(* Logix 5000 AddOnInstructionDefinition export Banner_QS18E_Param_v4; software revision 33.00 *)

TYPE Banner_IOL_Port_v4 :   // UDT that has all of the data items necessary to communicate with a specific Port on a IO-Link Master
STRUCT
   Port_Controlled : INT;   // Each bit represents a port on an IO-Link Master. Set to 1 to tell AOI to control that port.
   Port_Activate : INT;   // Each bit represents a port on an IO-Link Master. When ON that port will process any commands in queue.
   Port_Read : INT;   // Each bit represents a port on an IO-Link Master. Used to determine when device AOI has requested a Read command.
   Port_Write : INT;   // Each bit represents a port on an IO-Link Master. Used to determine when device AOI has requested a Write command.
   Port_RW_Complete : INT;   // Each bit represents a port on an IO-Link Master. Tells device AOI that Read or Write request has been completed.
   Port_Device_Read : INT;
   Data_Transfer : SINT[190];   // Array to transfer data from IO-Master to device AOIs.
END_STRUCT
END_TYPE

TYPE Banner_QS18E_1_v4 :   // Parameters for D, DV, LP, CV, and FP type sensors.
STRUCT
   Response_Speed : SINT;   // 0 = High Speed, 1 = Standard, 2 = Robust.
   Polarity_of_Pins_2_and_4 : SINT;   // 0 = Push Pull, 1 = PNP, 2 = NPN.
   Pin_2_Config : SINT;   // 0 = Deactivated, 1 = Pin 2 Emitter Enable, 2 = Pin 2 Emitter Disable, 3 = Remote Input, 4 = Detection Output, 5 = Complimentary Output, 6 = Normally Closed Health, 7 = Normally Open Health, 8 = Normally Closed Marginal, 9 = Normally Open Marginal.
   Process_Data_Input_Config : SINT;   // 0 = 5 and Signal, 1 = 5 and Count, 2 = 5 and Duration, 3 = 5 and Events per Minute.
   Marginal_Mode : SINT;   // 0 = Marginal Disabled, 1 = Marginal Auto, 2 = Marginal User.
   User_Marginal_Light : INT;   // 0 to 1000. User defined threshold.
   User_Marginal_Dark : INT;   // 0 to 1000. User defined threshold.
   LED_Power : SINT;   // 0 = Auto, 1 = Min Power, 2 = Power 2, 3 = Power 3, 4 = Power 4, 5 = Power 5, 6 = Max Power.
END_STRUCT
END_TYPE

TYPE Banner_QS18E_2_v4 :   // Parameters for EV and E type sensors
STRUCT
   Polarity_of_Pins_2_and_4 : SINT;   // 0 = Push Pull, 1 = PNP, 2 = NPN.
   Pin_2_Config : SINT;   // 0 = Deactivated, 1 = Pin 2 Emitter Enable, 2 = Pin 2 Emitter Disable, 3 = Remote Input, 4 = Detection Output, 5 = Complimentary Output, 6 = Normally Closed Health, 7 = Normally Open Health, 8 = Normally Closed Marginal, 9 = Normally Open Marginal.
   Frequency_Selection : SINT;   // 0 = High Speed, 1 = A, 2 = B, 3 = C.
   Power_Level : SINT;   // 0 to 5. Example: 5 = Power Level 5.
   Pushbutton_Lockout : SINT;   // 0 = Unlocked, 1 = Locked.
END_STRUCT
END_TYPE

TYPE Banner_QS18E_3_v4 :   // Parameters for RV and R type sensors
STRUCT
   Polarity_of_Pins_2_and_4 : SINT;   // 0 = Push Pull, 1 = PNP, 2 = NPN.
   Pin_2_Config : SINT;   // 0 = Deactivated, 1 = Pin 2 Emitter Enable, 2 = Pin 2 Emitter Disable, 3 = Remote Input, 4 = Detection Output, 5 = Complimentary Output, 6 = Normally Closed Health, 7 = Normally Open Health, 8 = Normally Closed Marginal, 9 = Normally Open Marginal.
   Process_Data_Input_Config : SINT;   // 0 = 5 and Signal, 1 = 5 and Count, 2 = 5 and Duration, 3 = 5 and Events per Minute.
   Marginal_Mode : SINT;   // 0 = Marginal Disabled, 1 = Marginal Auto, 2 = Marginal User.
   User_Marginal_Light : INT;   // 0 to 1000. User defined threshold.
   User_Marginal_Dark : INT;   // 0 to 1000. User defined threshold.
   Frequency_Selection : SINT;   // 0 = High Speed, 1 = A, 2 = B, 3 = C.
   IOL_Filter_Time : INT;   // Time in ms to average IOL process data measurement between updates.
   Gain : SINT;   // 0 = Auto - Teach, 1 = Auto - Run, 2 = Low Gain, 3 = Mid Gain, 4 = High Gain.
   Pushbutton_Lockout : SINT;   // 0 = Unlocked, 1 = Locked.
END_STRUCT
END_TYPE

TYPE Banner_QS18E_RD_v4 :   // UDT that stores the Write Data for a QS18E.
STRUCT
   Master_Cycle_Time : INT;
   Min_Cycle_Time : INT;
   M_Sequence_Capability : INT;
   IO_Link_Version_ID : INT;
   Process_Data_Input_Length : INT;
   Process_Data_Output_Length : INT;
   Combined_Vendor_ID : DINT;   // IO-Link Vendor ID
   Vendor_ID1 : INT;
   Vendor_ID2 : INT;
   Combined_Device_ID : DINT;   // IO-Link Device ID
   Device_ID1 : INT;
   Device_ID2 : INT;
   Device_ID3 : INT;
   Serial_Number : STRING;
   All_Time_Run_Time : DINT;   // Read only counter that tracks the total time sensor has been running since manufacture. Value in Hours.
   Quality_of_Health : INT;
   Normalized_Signal_Strength : INT;
   Quality_of_Teach : INT;
   Health_Lower_Limit : INT;
   Health_Upper_Limit : INT;
   SP2_Lower_Sensing_Threshold : INT;
   SP2_Upper_Sensing_Threshold : INT;
   SP1_Lower_Sensing_Threshold : INT;
   SP1_Upper_Sensing_Threshold : INT;
   Sensor_Operationl_Mode : INT;
   Output_Event_Count : DINT;
   Output_Event_Duration : DINT;
   Output_Event_Frequency : DINT;
   Active_Margninal_Light_Threshold : DINT;
   Active_Marginal_Dark_Threshold : DINT;
   Sigal : DINT;   // Only available for Sensor Type 3. Raw ADC Signal value.
END_STRUCT
END_TYPE

TYPE Banner_QS18E_v4 :   // All of the parameters for a QS18E.
STRUCT
   Initial_Global_Read : BOOL;   // Determines if all of the IO-Link data has been read into the PLC yet
   Command : INT;   // Value placed in here will activate a read or write to a specifc IO-Link Index
   Read_Data : Banner_QS18E_RD_v4;   // Read Only Data
   Write_Data : Banner_QS18E_WD_v4;   // Write Data
   Archive : Banner_QS18E_WD_v4;   // Archive Data
   Reset : BOOL;   // Resets AOI. This will force a complete parameter read of the sensor.
END_STRUCT
END_TYPE

TYPE Banner_QS18E_WD_v4 :   // UDT that stores the Write Data for a QS18E.
STRUCT
   System_Command : INT;   // See IODD file for list of commands that can be activated via the System Command interface
   Parameter_Access_Lock : SINT;   // Write access to all parameters is prohibited while value is 1. Only this parameter can be adjusted when value is 1.
   Data_Storage_Lock : SINT;   // Automatic data storage is disabled when this value is equal to 1. Read access is not affected.
   Local_Parameterization_Lock : SINT;   // Parameterization via local control elements on device is disabled.
   Local_User_Interface_Lock : SINT;   // Operation of local user interface is disabled.
   BDC1_Swithpoint_Logic : INT;   // 0 = Light Operate, 1 = Dark Operate
   BDC1_BDC_Mode : INT;   // 1 = 1-Pt BGS, 128 = 2-Pt, 129 = Dynamic, 130 = Window or FGS, 131 = Dual
   BDC1_Hysteresis : DINT;   // Should always be 0
   Marginal_Signal_Delay : DINT;   // 0 to 60000. Millisecond value
   User_Health_Setting : INT;   // 0 to 90
   Offset_Percent : INT;   // 0 = Min, 1 = 10%, 2 = 15%, 3 = 20%, 4 = 25%, 5 = 30%, 6 = 40%, 7 = 50%, 8 = 100%, 9 = 200%.
   Auto_Compensaton : INT;   // 0=Disabled, 1=Enabled
   Delay_Timer_2 : DINT;   // 0 to 90000 ms
   Delay_Timer_1 : DINT;   // 0 to 90000 ms
   Delay_Mode : INT;   // 0=Disabled, 1=On Off Delay, 2=On One Shot, 3=Off One Shot
   Resettable_Run_Time : DINT;
   Type_1_Data : Banner_QS18E_1_v4;   // Data for a D, DV, Lp, VC, or FP QS18E type sensor.
   Type_2_Data : Banner_QS18E_2_v4;   // Data for a E or EV QS18E type sensor.
   Type_3_Data : Banner_QS18E_3_v4;   // Data for a R or RV QS18E type sensor.
   All_Time_Run_Time_Event_Time : DINT;
   Resettable_Run_Time_Event_Time : DINT;
END_STRUCT
END_TYPE

ADD_ON_INSTRUCTION Banner_QS18E_Param_v4   (* revision 4.0, vendor Banner Engineering *)
// AOI to read and write parameter data to an IO-Link QS18E.
// Revision note:
// Updated for QS18 Emitter and Receiver.
VAR_IN_OUT
   QS18E : Banner_QS18E_v4; {required}
   Port_Data : Banner_IOL_Port_v4; {required}
END_VAR
VAR_INPUT
   Port : DINT; {required}
   Sensor_Type : DINT; {required}   // 1 = D, DV, LP, CV, & FP models, 2 = EV or E models, 3 = RV or R models.
END_VAR
VAR
   Local_Control : DINT; {access None}
   Global_Read_Command_Value : INT; {access None}
   Global_Write_Command_Value : INT; {access None}
   Command_Being_Processed : BOOL; {access None}
   Update_Archive : BOOL; {access None}
   Index_Write_Inprocess : INT; {access None}
   Index_Write_Control : INT; {access None}
   Inprocess_Index : DINT; {access None}
END_VAR

ROUTINE Logic   (* ladder *)
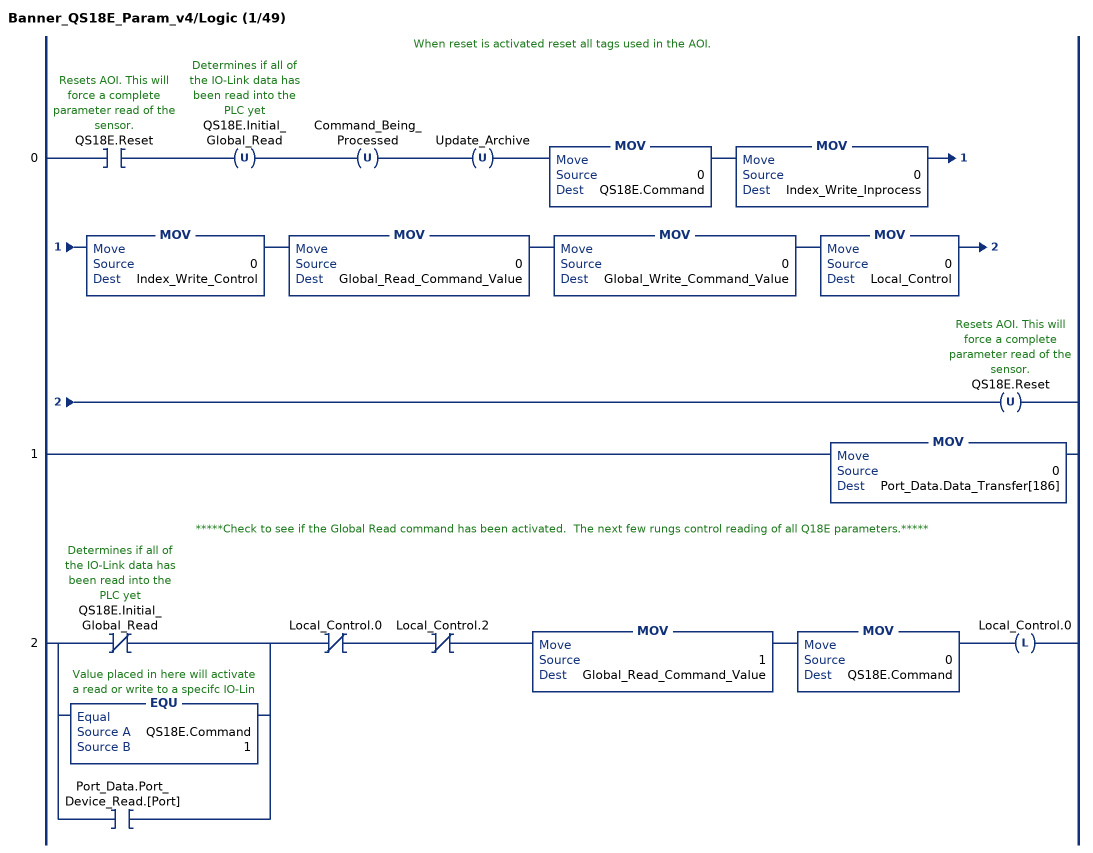
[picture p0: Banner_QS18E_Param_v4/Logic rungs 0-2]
   // When reset is activated reset all tags used in the AOI.
   0: XIC(QS18E.Reset)OTU(QS18E.Initial_Global_Read)OTU(Command_Being_Processed)OTU(Update_Archive)MOV(0,QS18E.Command)MOV(0,Index_Write_Inprocess)MOV(0,Index_Write_Control)MOV(0,Global_Read_Command_Value)MOV(0,Global_Write_Command_Value)MOV(0,Local_Control)OTU(QS18E.Reset);
   1: MOV(0,Port_Data.Data_Transfer[186]);
   // *****Check to see if the Global Read command has been activated.  The next few rungs control reading of all Q18E parameters.*****
   2: [XIO(QS18E.Initial_Global_Read) ,EQU(QS18E.Command,1) ,XIC(Port_Data.Port_Device_Read.[Port]) ]XIO(Local_Control.0)XIO(Local_Control.2)MOV(1,Global_Read_Command_Value)MOV(0,QS18E.Command)OTL(Local_Control.0);
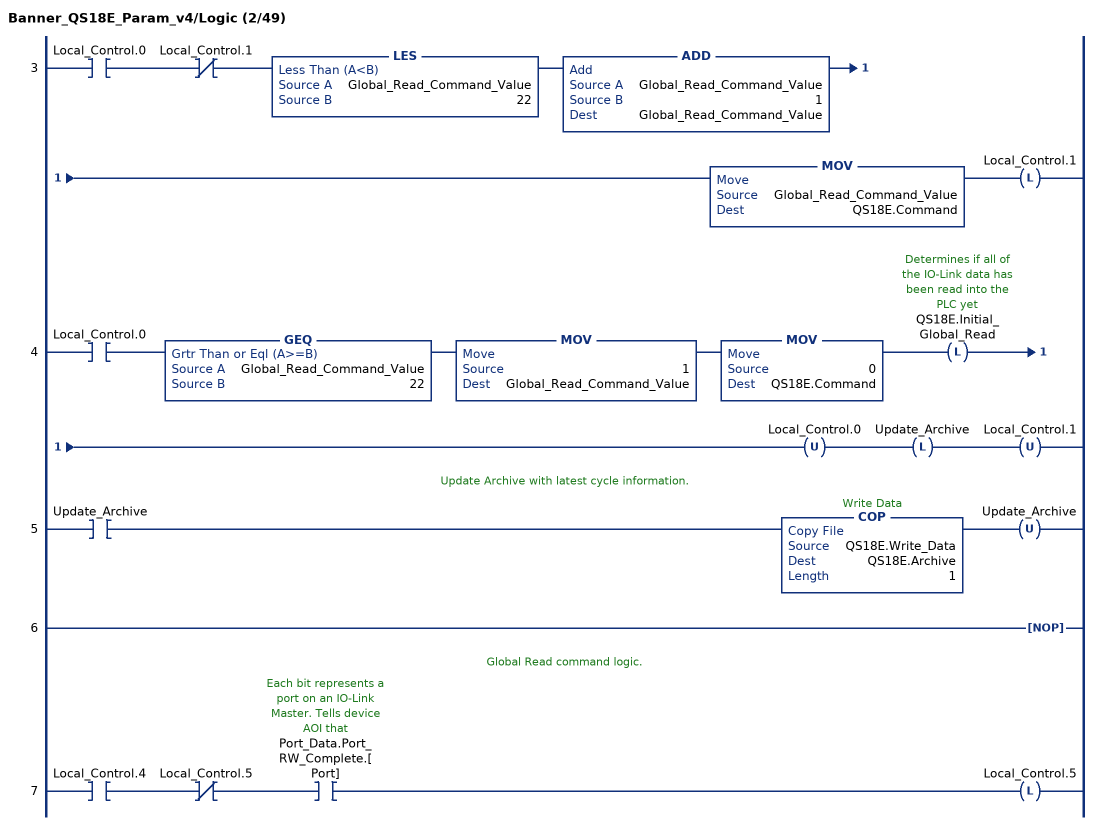
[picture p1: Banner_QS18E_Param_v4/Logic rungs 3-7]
   3: XIC(Local_Control.0)XIO(Local_Control.1)LES(Global_Read_Command_Value,22)ADD(Global_Read_Command_Value,1,Global_Read_Command_Value)MOV(Global_Read_Command_Value,QS18E.Command)OTL(Local_Control.1);
   4: XIC(Local_Control.0)GEQ(Global_Read_Command_Value,22)MOV(1,Global_Read_Command_Value)MOV(0,QS18E.Command)OTL(QS18E.Initial_Global_Read)OTU(Local_Control.0)OTL(Update_Archive)OTU(Local_Control.1);
   // Update Archive with latest cycle information.
   5: XIC(Update_Archive)COP(QS18E.Write_Data,QS18E.Archive,1)OTU(Update_Archive);
   6: NOP();
   // Global Read command logic.
   7: XIC(Local_Control.4)XIO(Local_Control.5)XIC(Port_Data.Port_RW_Complete.[Port])OTL(Local_Control.5);
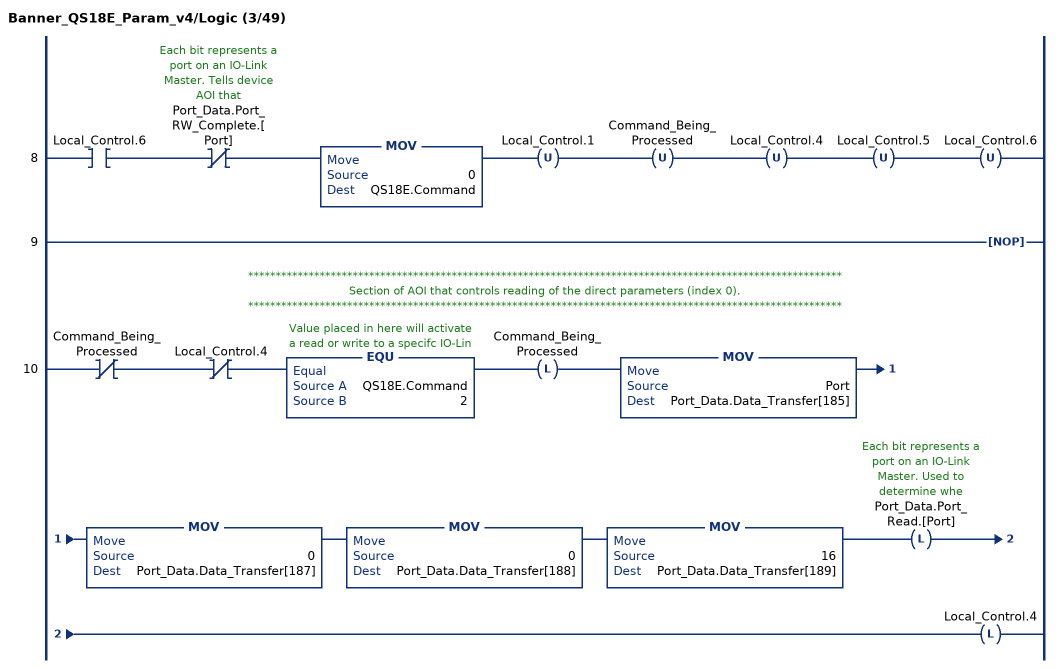
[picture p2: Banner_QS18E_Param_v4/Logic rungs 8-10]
   8: XIC(Local_Control.6)XIO(Port_Data.Port_RW_Complete.[Port])MOV(0,QS18E.Command)OTU(Local_Control.1)OTU(Command_Being_Processed)OTU(Local_Control.4)OTU(Local_Control.5)OTU(Local_Control.6);
   9: NOP();
   // ************************************************************************************************************
   // Section of AOI that controls reading of the direct parameters (index 0).
   // ************************************************************************************************************
   10: XIO(Command_Being_Processed)XIO(Local_Control.4)EQU(QS18E.Command,2)OTL(Command_Being_Processed)MOV(Port,Port_Data.Data_Transfer[185])MOV(0,Port_Data.Data_Transfer[187])MOV(0,Port_Data.Data_Transfer[188])MOV(16,Port_Data.Data_Transfer[189])OTL(Port_Data.Port_Read.[Port])OTL(Local_Control.4);
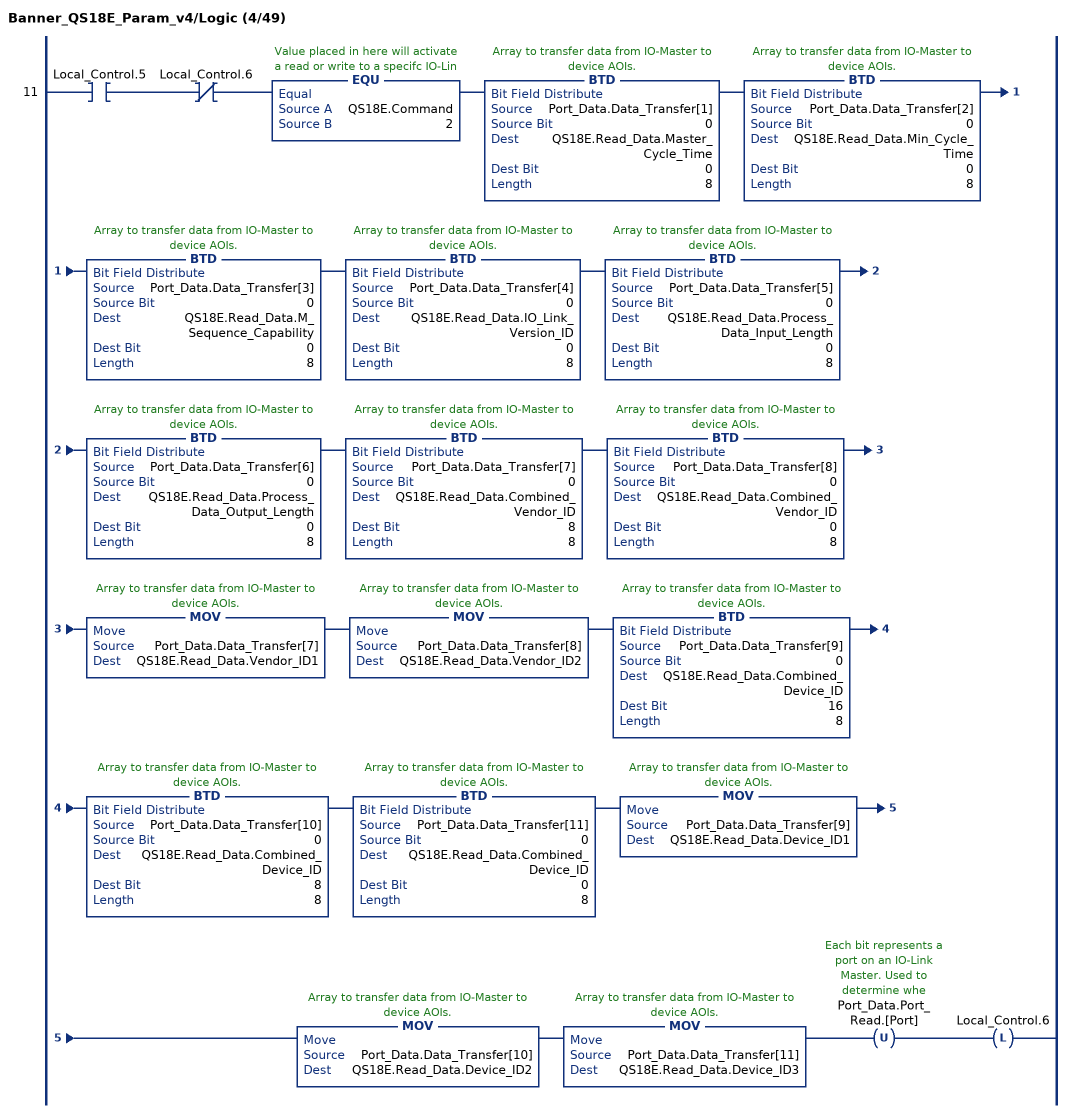
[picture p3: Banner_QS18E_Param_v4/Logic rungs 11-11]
   11: XIC(Local_Control.5)XIO(Local_Control.6)EQU(QS18E.Command,2)BTD(Port_Data.Data_Transfer[1],0,QS18E.Read_Data.Master_Cycle_Time,0,8)BTD(Port_Data.Data_Transfer[2],0,QS18E.Read_Data.Min_Cycle_Time,0,8)BTD(Port_Data.Data_Transfer[3],0,QS18E.Read_Data.M_Sequence_Capability,0,8)BTD(Port_Data.Data_Transfer[4],0,QS18E.Read_Data.IO_Link_Version_ID,0,8)BTD(Port_Data.Data_Transfer[5],0,QS18E.Read_Data.Process_Data_Input_Length,0,8)BTD(Port_Data.Data_Transfer[6],0,QS18E.Read_Data.Process_Data_Output_Length,0,8)BTD(Port_Data.Data_Transfer[7],0,QS18E.Read_Data.Combined_Vendor_ID,8,8)BTD(Port_Data.Data_Transfer[8],0,QS18E.Read_Data.Combined_Vendor_ID,0,8)MOV(Port_Data.Data_Transfer[7],QS18E.Read_Data.Vendor_ID1)MOV(Port_Data.Data_Transfer[8],QS18E.Read_Data.Vendor_ID2)BTD(Port_Data.Data_Transfer[9],0,QS18E.Read_Data.Combined_Device_ID,16,8)BTD(Port_Data.Data_Transfer[10],0,QS18E.Read_Data.Combined_Device_ID,8,8)BTD(Port_Data.Data_Transfer[11],0,QS18E.Read_Data.Combined_Device_ID,0,8)MOV(Port_Data.Data_Transfer[9],QS18E.Read_Data.Device_ID1)MOV(Port_Data.Data_Transfer[10],QS18E.Read_Data.Device_ID2)MOV(Port_Data.Data_Transfer[11],QS18E.Read_Data.Device_ID3)OTU(Port_Data.Port_Read.[Port])OTL(Local_Control.6);
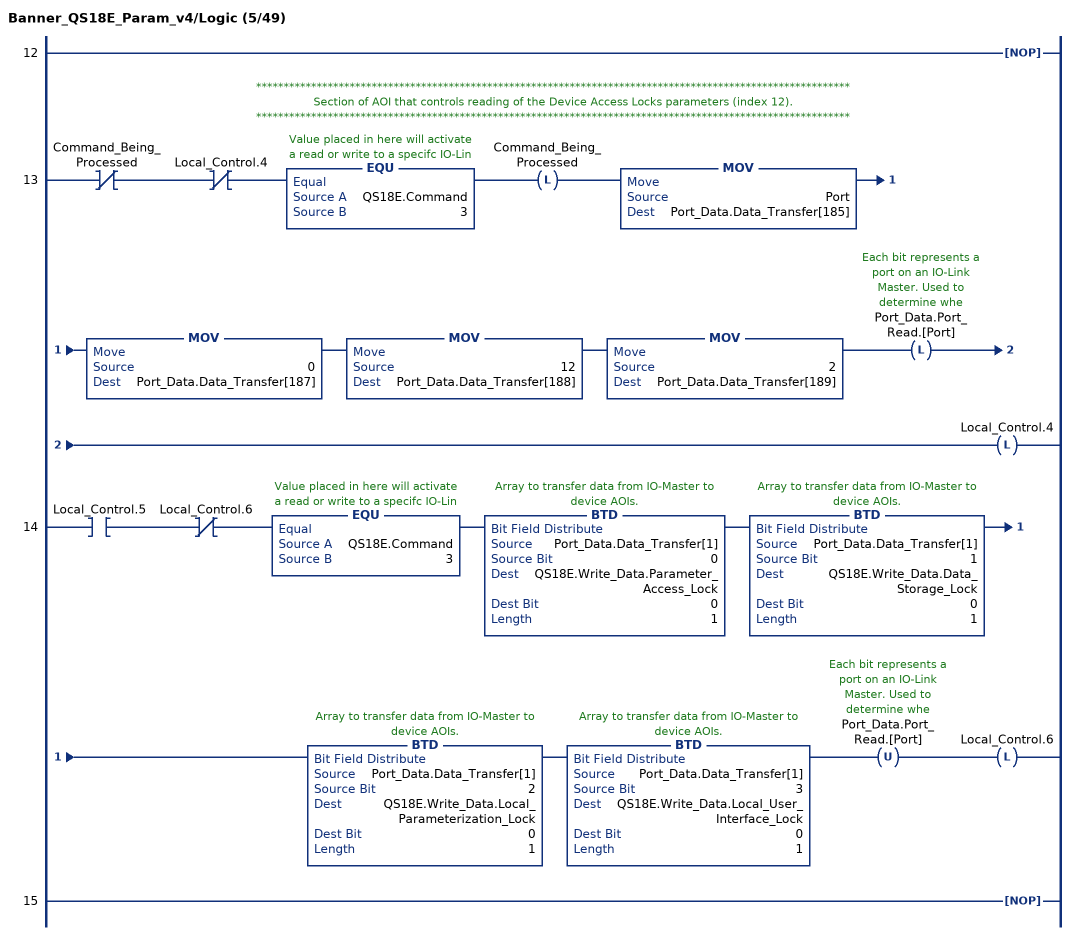
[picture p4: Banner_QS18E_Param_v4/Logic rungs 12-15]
   12: NOP();
   // ************************************************************************************************************
   // Section of AOI that controls reading of the Device Access Locks parameters (index 12).
   // ************************************************************************************************************
   13: XIO(Command_Being_Processed)XIO(Local_Control.4)EQU(QS18E.Command,3)OTL(Command_Being_Processed)MOV(Port,Port_Data.Data_Transfer[185])MOV(0,Port_Data.Data_Transfer[187])MOV(12,Port_Data.Data_Transfer[188])MOV(2,Port_Data.Data_Transfer[189])OTL(Port_Data.Port_Read.[Port])OTL(Local_Control.4);
   14: XIC(Local_Control.5)XIO(Local_Control.6)EQU(QS18E.Command,3)BTD(Port_Data.Data_Transfer[1],0,QS18E.Write_Data.Parameter_Access_Lock,0,1)BTD(Port_Data.Data_Transfer[1],1,QS18E.Write_Data.Data_Storage_Lock,0,1)BTD(Port_Data.Data_Transfer[1],2,QS18E.Write_Data.Local_Parameterization_Lock,0,1)BTD(Port_Data.Data_Transfer[1],3,QS18E.Write_Data.Local_User_Interface_Lock,0,1)OTU(Port_Data.Port_Read.[Port])OTL(Local_Control.6);
   15: NOP();
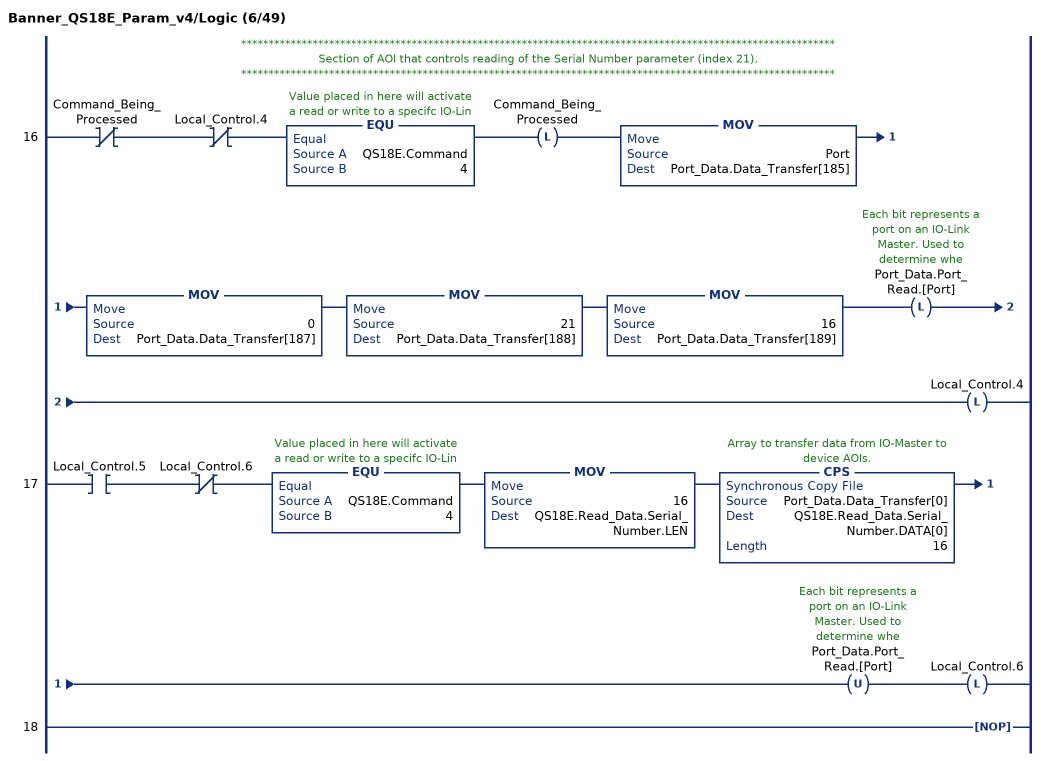
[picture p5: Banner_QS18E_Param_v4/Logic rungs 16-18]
   // ************************************************************************************************************
   // Section of AOI that controls reading of the Serial Number parameter (index 21).
   // ************************************************************************************************************
   16: XIO(Command_Being_Processed)XIO(Local_Control.4)EQU(QS18E.Command,4)OTL(Command_Being_Processed)MOV(Port,Port_Data.Data_Transfer[185])MOV(0,Port_Data.Data_Transfer[187])MOV(21,Port_Data.Data_Transfer[188])MOV(16,Port_Data.Data_Transfer[189])OTL(Port_Data.Port_Read.[Port])OTL(Local_Control.4);
   17: XIC(Local_Control.5)XIO(Local_Control.6)EQU(QS18E.Command,4)MOV(16,QS18E.Read_Data.Serial_Number.LEN)CPS(Port_Data.Data_Transfer[0],QS18E.Read_Data.Serial_Number.DATA[0],16)OTU(Port_Data.Port_Read.[Port])OTL(Local_Control.6);
   18: NOP();
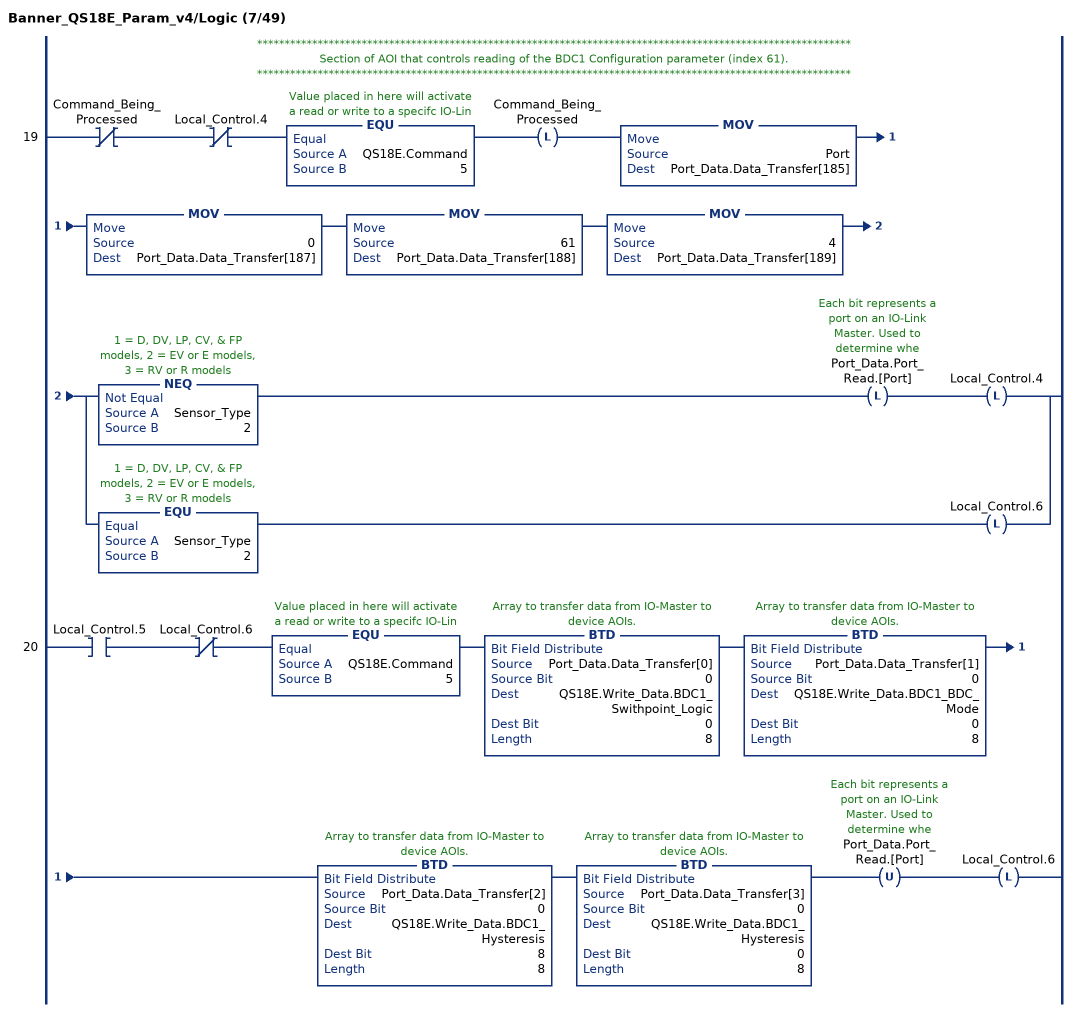
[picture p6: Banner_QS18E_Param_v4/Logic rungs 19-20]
   // ************************************************************************************************************
   // Section of AOI that controls reading of the BDC1 Configuration parameter (index 61).
   // ************************************************************************************************************
   19: XIO(Command_Being_Processed)XIO(Local_Control.4)EQU(QS18E.Command,5)OTL(Command_Being_Processed)MOV(Port,Port_Data.Data_Transfer[185])MOV(0,Port_Data.Data_Transfer[187])MOV(61,Port_Data.Data_Transfer[188])MOV(4,Port_Data.Data_Transfer[189])[NEQ(Sensor_Type,2) OTL(Port_Data.Port_Read.[Port]) OTL(Local_Control.4) ,EQU(Sensor_Type,2) OTL(Local_Control.6) ];
   20: XIC(Local_Control.5)XIO(Local_Control.6)EQU(QS18E.Command,5)BTD(Port_Data.Data_Transfer[0],0,QS18E.Write_Data.BDC1_Swithpoint_Logic,0,8)BTD(Port_Data.Data_Transfer[1],0,QS18E.Write_Data.BDC1_BDC_Mode,0,8)BTD(Port_Data.Data_Transfer[2],0,QS18E.Write_Data.BDC1_Hysteresis,8,8)BTD(Port_Data.Data_Transfer[3],0,QS18E.Write_Data.BDC1_Hysteresis,0,8)OTU(Port_Data.Port_Read.[Port])OTL(Local_Control.6);
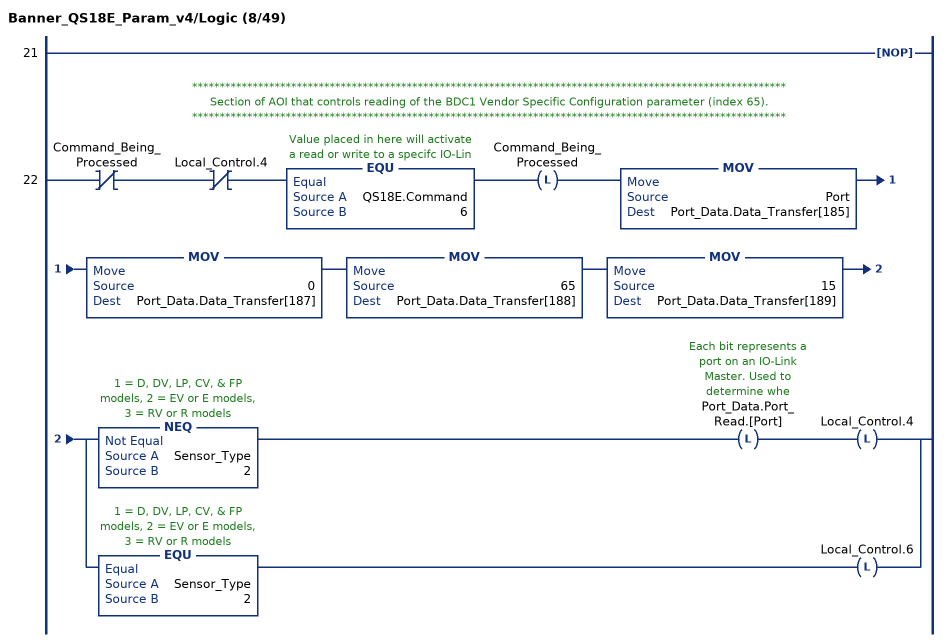
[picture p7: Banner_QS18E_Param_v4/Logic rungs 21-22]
   21: NOP();
   // ************************************************************************************************************
   // Section of AOI that controls reading of the BDC1 Vendor Specific Configuration parameter (index 65).
   // ************************************************************************************************************
   22: XIO(Command_Being_Processed)XIO(Local_Control.4)EQU(QS18E.Command,6)OTL(Command_Being_Processed)MOV(Port,Port_Data.Data_Transfer[185])MOV(0,Port_Data.Data_Transfer[187])MOV(65,Port_Data.Data_Transfer[188])MOV(15,Port_Data.Data_Transfer[189])[NEQ(Sensor_Type,2) OTL(Port_Data.Port_Read.[Port]) OTL(Local_Control.4) ,EQU(Sensor_Type,2) OTL(Local_Control.6) ];
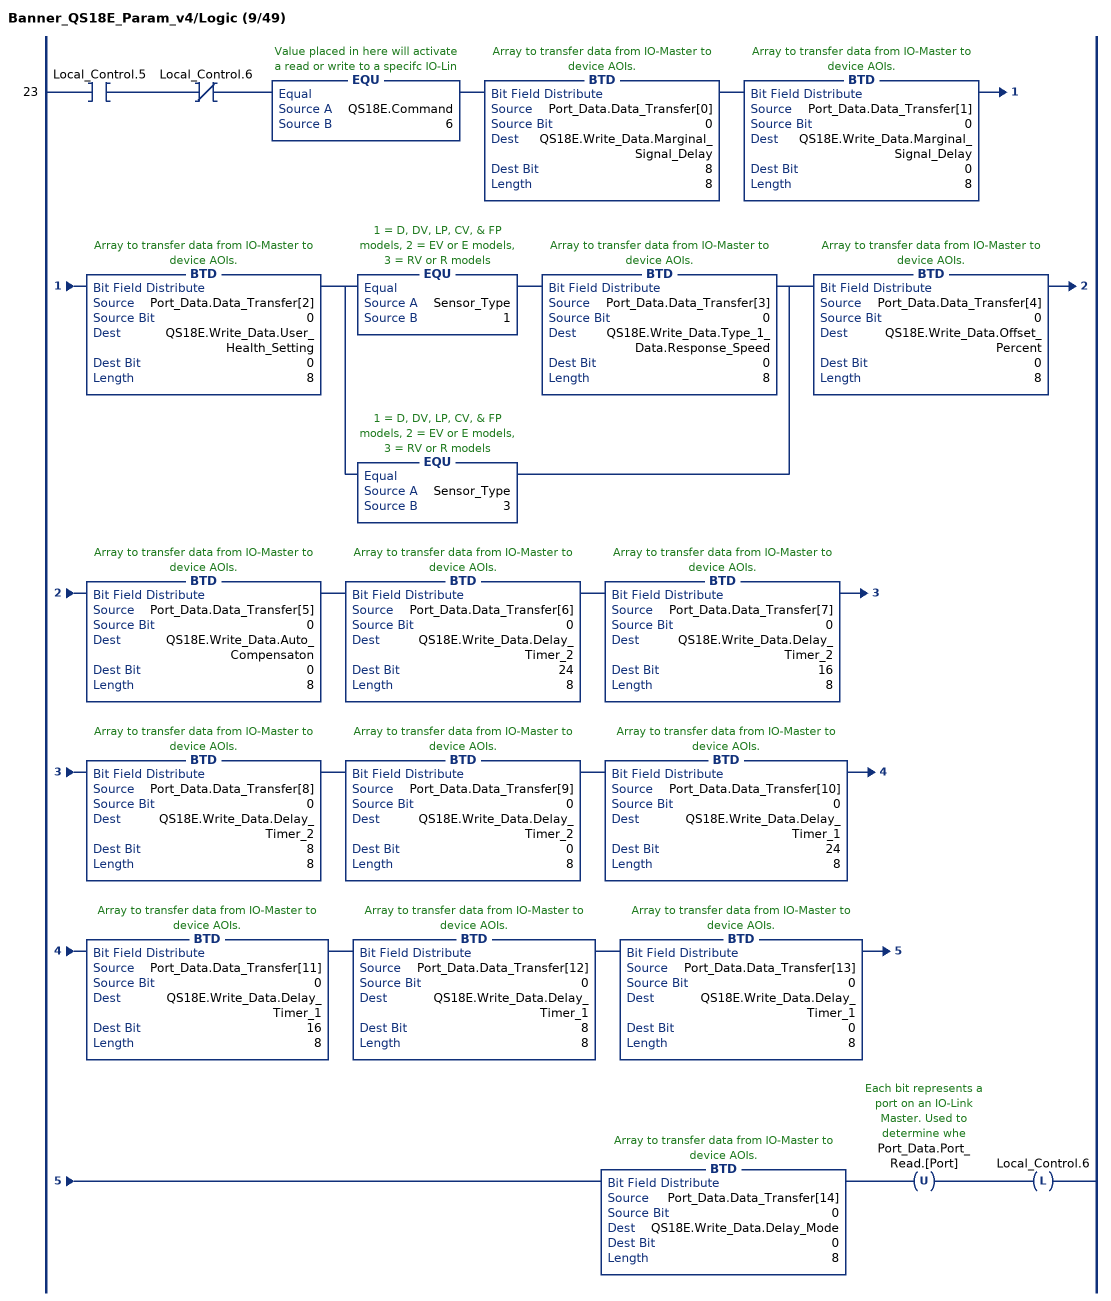
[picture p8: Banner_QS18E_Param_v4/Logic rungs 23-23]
   23: XIC(Local_Control.5)XIO(Local_Control.6)EQU(QS18E.Command,6)BTD(Port_Data.Data_Transfer[0],0,QS18E.Write_Data.Marginal_Signal_Delay,8,8)BTD(Port_Data.Data_Transfer[1],0,QS18E.Write_Data.Marginal_Signal_Delay,0,8)BTD(Port_Data.Data_Transfer[2],0,QS18E.Write_Data.User_Health_Setting,0,8)[EQU(Sensor_Type,1) BTD(Port_Data.Data_Transfer[3],0,QS18E.Write_Data.Type_1_Data.Response_Speed,0,8) ,EQU(Sensor_Type,3) ]BTD(Port_Data.Data_Transfer[4],0,QS18E.Write_Data.Offset_Percent,0,8)BTD(Port_Data.Data_Transfer[5],0,QS18E.Write_Data.Auto_Compensaton,0,8)BTD(Port_Data.Data_Transfer[6],0,QS18E.Write_Data.Delay_Timer_2,24,8)BTD(Port_Data.Data_Transfer[7],0,QS18E.Write_Data.Delay_Timer_2,16,8)BTD(Port_Data.Data_Transfer[8],0,QS18E.Write_Data.Delay_Timer_2,8,8)BTD(Port_Data.Data_Transfer[9],0,QS18E.Write_Data.Delay_Timer_2,0,8)BTD(Port_Data.Data_Transfer[10],0,QS18E.Write_Data.Delay_Timer_1,24,8)BTD(Port_Data.Data_Transfer[11],0,QS18E.Write_Data.Delay_Timer_1,16,8)BTD(Port_Data.Data_Transfer[12],0,QS18E.Write_Data.Delay_Timer_1,8,8)BTD(Port_Data.Data_Transfer[13],0,QS18E.Write_Data.Delay_Timer_1,0,8)BTD(Port_Data.Data_Transfer[14],0,QS18E.Write_Data.Delay_Mode,0,8)OTU(Port_Data.Port_Read.[Port])OTL(Local_Control.6);
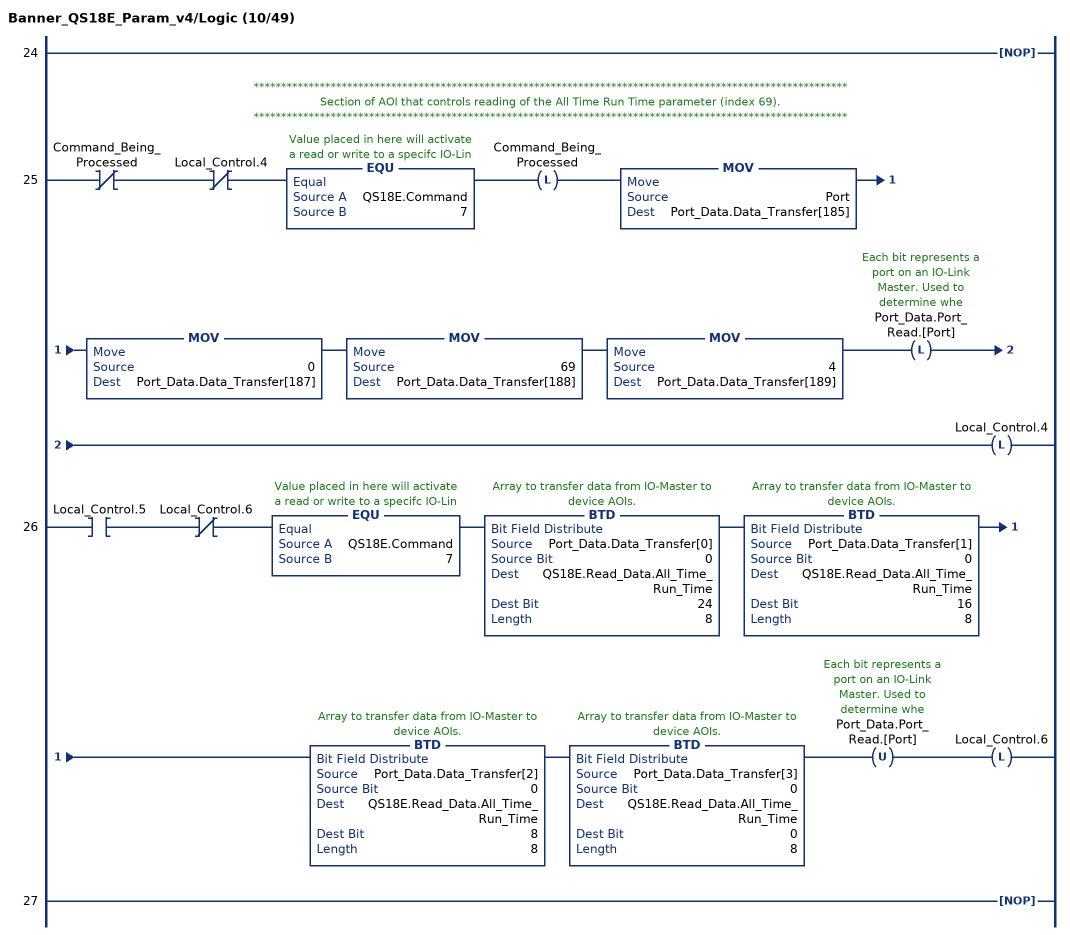
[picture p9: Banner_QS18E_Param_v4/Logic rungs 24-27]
   24: NOP();
   // ************************************************************************************************************
   // Section of AOI that controls reading of the All Time Run Time parameter (index 69).
   // ************************************************************************************************************
   25: XIO(Command_Being_Processed)XIO(Local_Control.4)EQU(QS18E.Command,7)OTL(Command_Being_Processed)MOV(Port,Port_Data.Data_Transfer[185])MOV(0,Port_Data.Data_Transfer[187])MOV(69,Port_Data.Data_Transfer[188])MOV(4,Port_Data.Data_Transfer[189])OTL(Port_Data.Port_Read.[Port])OTL(Local_Control.4);
   26: XIC(Local_Control.5)XIO(Local_Control.6)EQU(QS18E.Command,7)BTD(Port_Data.Data_Transfer[0],0,QS18E.Read_Data.All_Time_Run_Time,24,8)BTD(Port_Data.Data_Transfer[1],0,QS18E.Read_Data.All_Time_Run_Time,16,8)BTD(Port_Data.Data_Transfer[2],0,QS18E.Read_Data.All_Time_Run_Time,8,8)BTD(Port_Data.Data_Transfer[3],0,QS18E.Read_Data.All_Time_Run_Time,0,8)OTU(Port_Data.Port_Read.[Port])OTL(Local_Control.6);
   27: NOP();
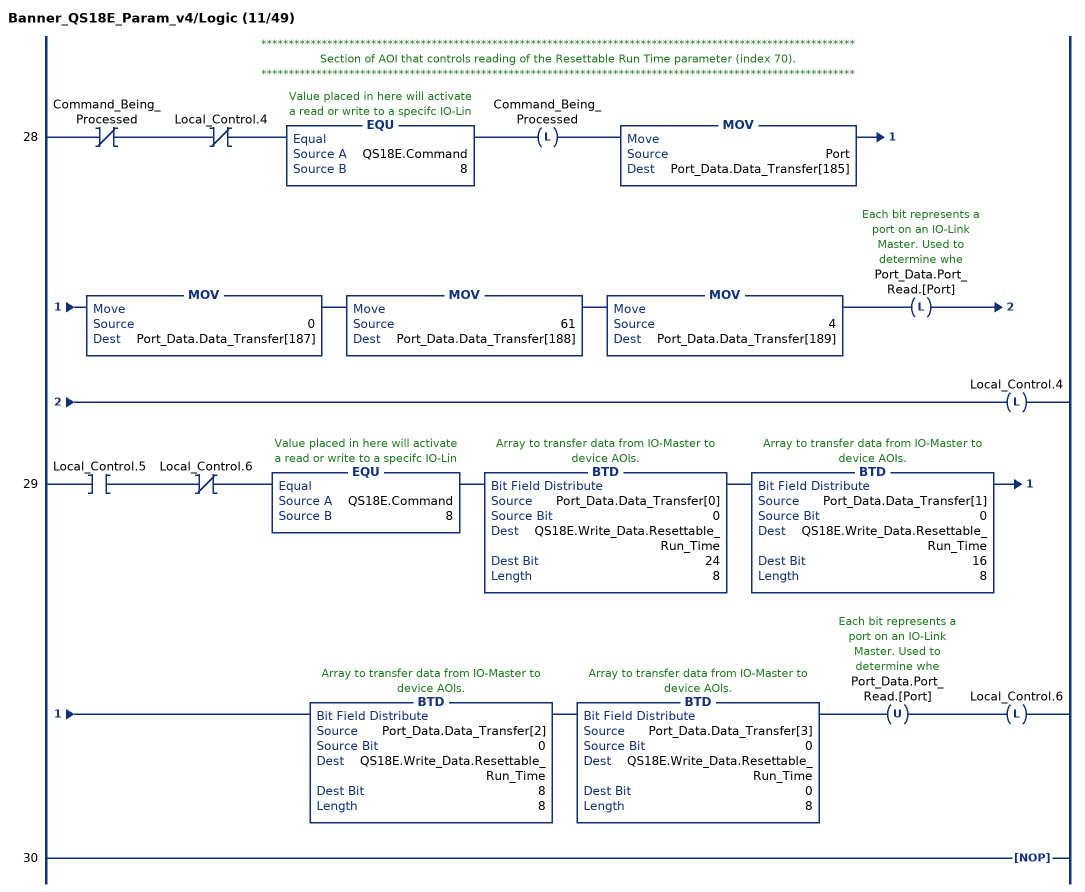
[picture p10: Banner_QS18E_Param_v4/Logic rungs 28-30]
   // ************************************************************************************************************
   // Section of AOI that controls reading of the Resettable Run Time parameter (index 70).
   // ************************************************************************************************************
   28: XIO(Command_Being_Processed)XIO(Local_Control.4)EQU(QS18E.Command,8)OTL(Command_Being_Processed)MOV(Port,Port_Data.Data_Transfer[185])MOV(0,Port_Data.Data_Transfer[187])MOV(61,Port_Data.Data_Transfer[188])MOV(4,Port_Data.Data_Transfer[189])OTL(Port_Data.Port_Read.[Port])OTL(Local_Control.4);
   29: XIC(Local_Control.5)XIO(Local_Control.6)EQU(QS18E.Command,8)BTD(Port_Data.Data_Transfer[0],0,QS18E.Write_Data.Resettable_Run_Time,24,8)BTD(Port_Data.Data_Transfer[1],0,QS18E.Write_Data.Resettable_Run_Time,16,8)BTD(Port_Data.Data_Transfer[2],0,QS18E.Write_Data.Resettable_Run_Time,8,8)BTD(Port_Data.Data_Transfer[3],0,QS18E.Write_Data.Resettable_Run_Time,0,8)OTU(Port_Data.Port_Read.[Port])OTL(Local_Control.6);
   30: NOP();
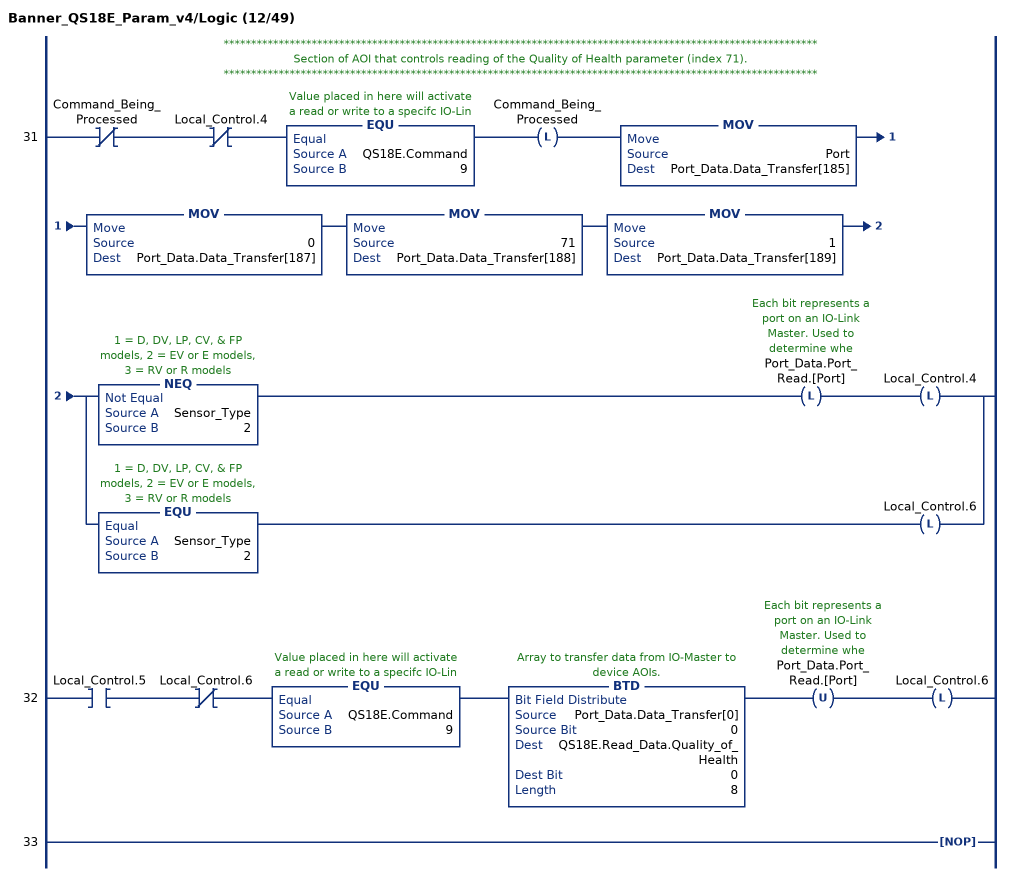
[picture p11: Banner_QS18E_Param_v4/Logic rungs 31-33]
   // ************************************************************************************************************
   // Section of AOI that controls reading of the Quality of Health parameter (index 71).
   // ************************************************************************************************************
   31: XIO(Command_Being_Processed)XIO(Local_Control.4)EQU(QS18E.Command,9)OTL(Command_Being_Processed)MOV(Port,Port_Data.Data_Transfer[185])MOV(0,Port_Data.Data_Transfer[187])MOV(71,Port_Data.Data_Transfer[188])MOV(1,Port_Data.Data_Transfer[189])[NEQ(Sensor_Type,2) OTL(Port_Data.Port_Read.[Port]) OTL(Local_Control.4) ,EQU(Sensor_Type,2) OTL(Local_Control.6) ];
   32: XIC(Local_Control.5)XIO(Local_Control.6)EQU(QS18E.Command,9)BTD(Port_Data.Data_Transfer[0],0,QS18E.Read_Data.Quality_of_Health,0,8)OTU(Port_Data.Port_Read.[Port])OTL(Local_Control.6);
   33: NOP();
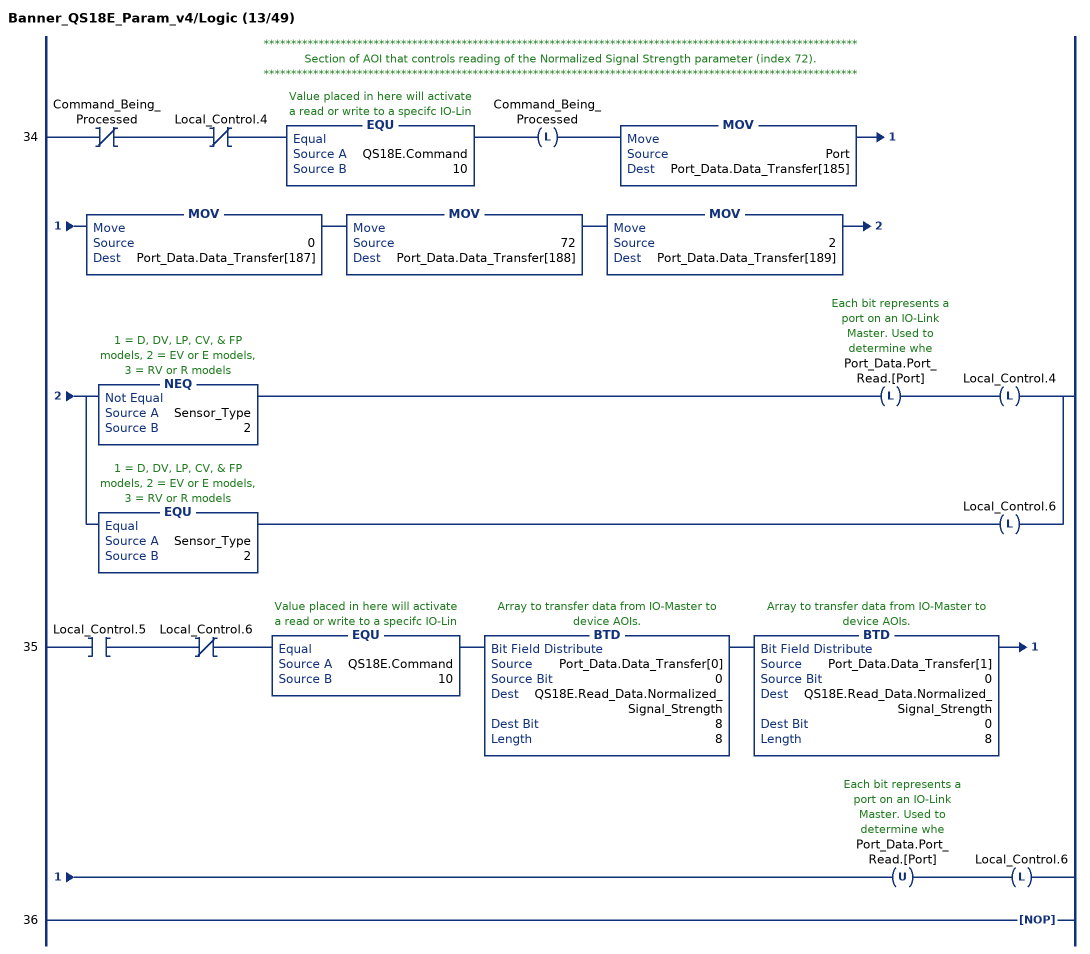
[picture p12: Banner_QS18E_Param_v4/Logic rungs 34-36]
   // ************************************************************************************************************
   // Section of AOI that controls reading of the Normalized Signal Strength parameter (index 72).
   // ************************************************************************************************************
   34: XIO(Command_Being_Processed)XIO(Local_Control.4)EQU(QS18E.Command,10)OTL(Command_Being_Processed)MOV(Port,Port_Data.Data_Transfer[185])MOV(0,Port_Data.Data_Transfer[187])MOV(72,Port_Data.Data_Transfer[188])MOV(2,Port_Data.Data_Transfer[189])[NEQ(Sensor_Type,2) OTL(Port_Data.Port_Read.[Port]) OTL(Local_Control.4) ,EQU(Sensor_Type,2) OTL(Local_Control.6) ];
   35: XIC(Local_Control.5)XIO(Local_Control.6)EQU(QS18E.Command,10)BTD(Port_Data.Data_Transfer[0],0,QS18E.Read_Data.Normalized_Signal_Strength,8,8)BTD(Port_Data.Data_Transfer[1],0,QS18E.Read_Data.Normalized_Signal_Strength,0,8)OTU(Port_Data.Port_Read.[Port])OTL(Local_Control.6);
   36: NOP();
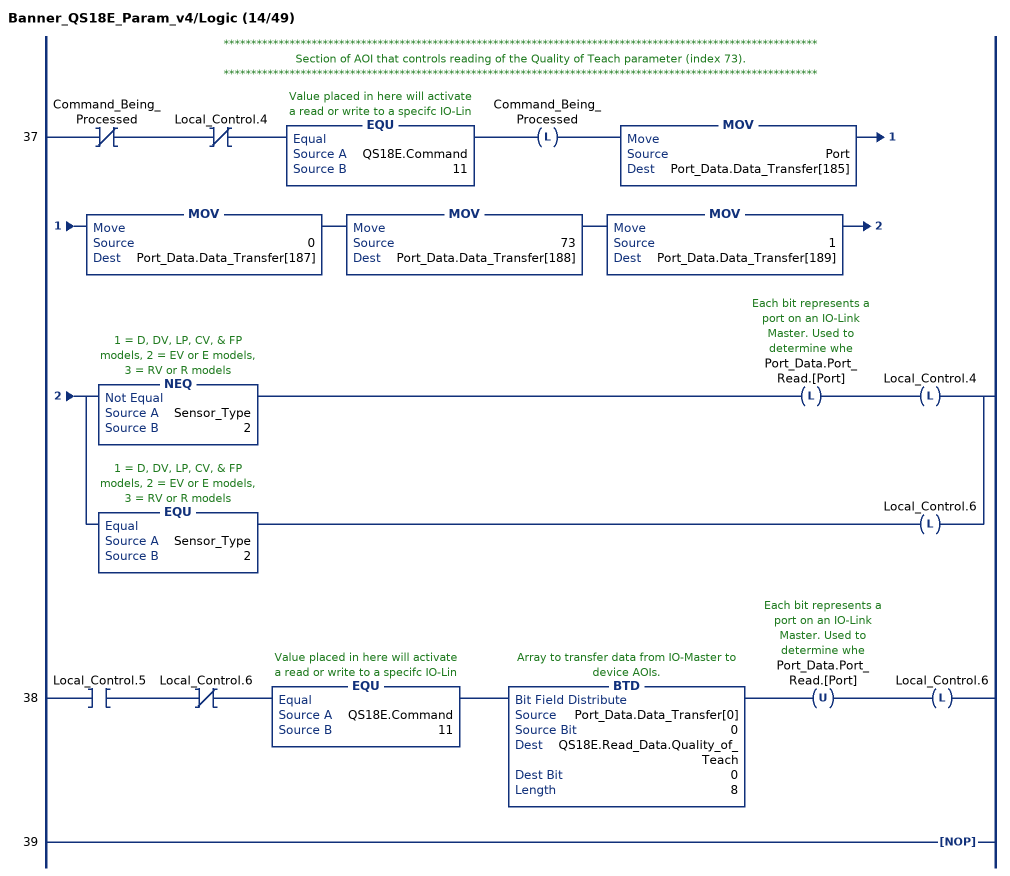
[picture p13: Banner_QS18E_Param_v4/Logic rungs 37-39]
   // ************************************************************************************************************
   // Section of AOI that controls reading of the Quality of Teach parameter (index 73).
   // ************************************************************************************************************
   37: XIO(Command_Being_Processed)XIO(Local_Control.4)EQU(QS18E.Command,11)OTL(Command_Being_Processed)MOV(Port,Port_Data.Data_Transfer[185])MOV(0,Port_Data.Data_Transfer[187])MOV(73,Port_Data.Data_Transfer[188])MOV(1,Port_Data.Data_Transfer[189])[NEQ(Sensor_Type,2) OTL(Port_Data.Port_Read.[Port]) OTL(Local_Control.4) ,EQU(Sensor_Type,2) OTL(Local_Control.6) ];
   38: XIC(Local_Control.5)XIO(Local_Control.6)EQU(QS18E.Command,11)BTD(Port_Data.Data_Transfer[0],0,QS18E.Read_Data.Quality_of_Teach,0,8)OTU(Port_Data.Port_Read.[Port])OTL(Local_Control.6);
   39: NOP();
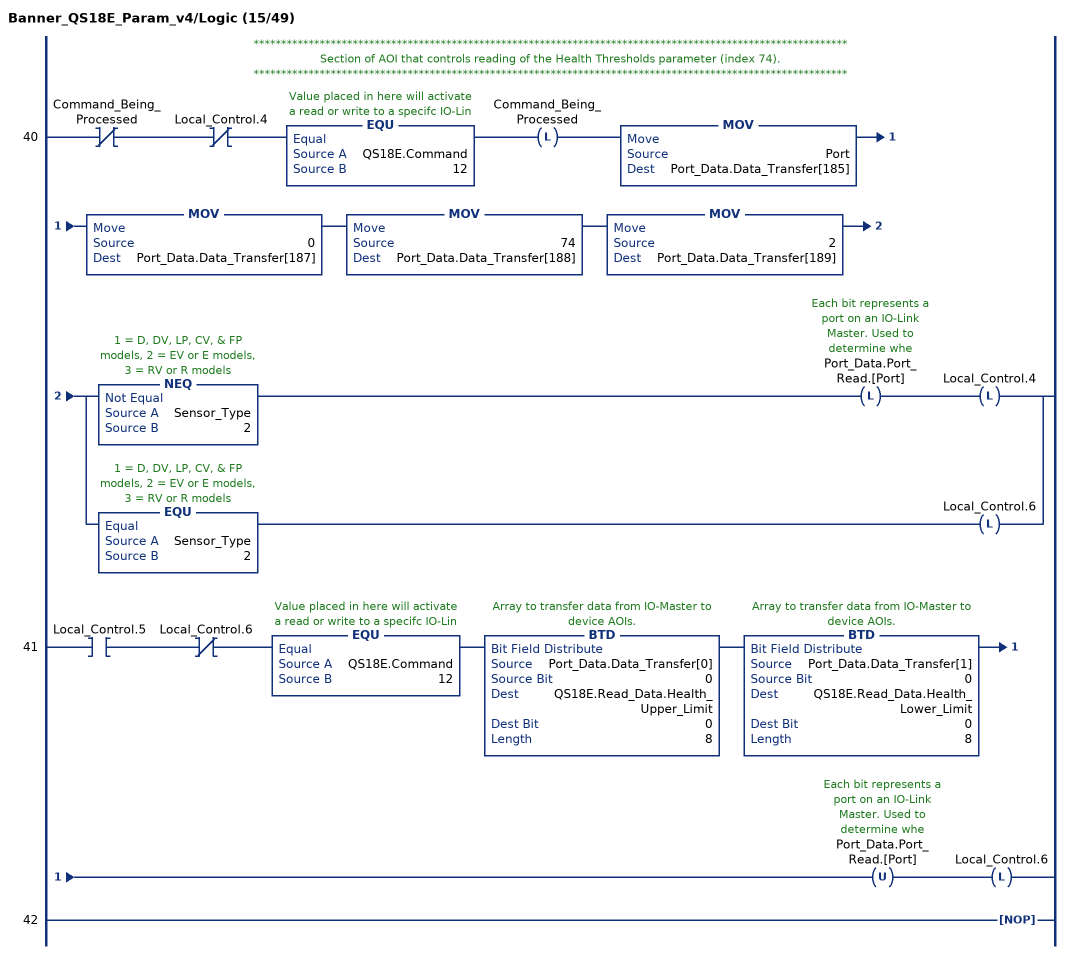
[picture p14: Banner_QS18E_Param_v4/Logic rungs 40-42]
   // ************************************************************************************************************
   // Section of AOI that controls reading of the Health Thresholds parameter (index 74).
   // ************************************************************************************************************
   40: XIO(Command_Being_Processed)XIO(Local_Control.4)EQU(QS18E.Command,12)OTL(Command_Being_Processed)MOV(Port,Port_Data.Data_Transfer[185])MOV(0,Port_Data.Data_Transfer[187])MOV(74,Port_Data.Data_Transfer[188])MOV(2,Port_Data.Data_Transfer[189])[NEQ(Sensor_Type,2) OTL(Port_Data.Port_Read.[Port]) OTL(Local_Control.4) ,EQU(Sensor_Type,2) OTL(Local_Control.6) ];
   41: XIC(Local_Control.5)XIO(Local_Control.6)EQU(QS18E.Command,12)BTD(Port_Data.Data_Transfer[0],0,QS18E.Read_Data.Health_Upper_Limit,0,8)BTD(Port_Data.Data_Transfer[1],0,QS18E.Read_Data.Health_Lower_Limit,0,8)OTU(Port_Data.Port_Read.[Port])OTL(Local_Control.6);
   42: NOP();
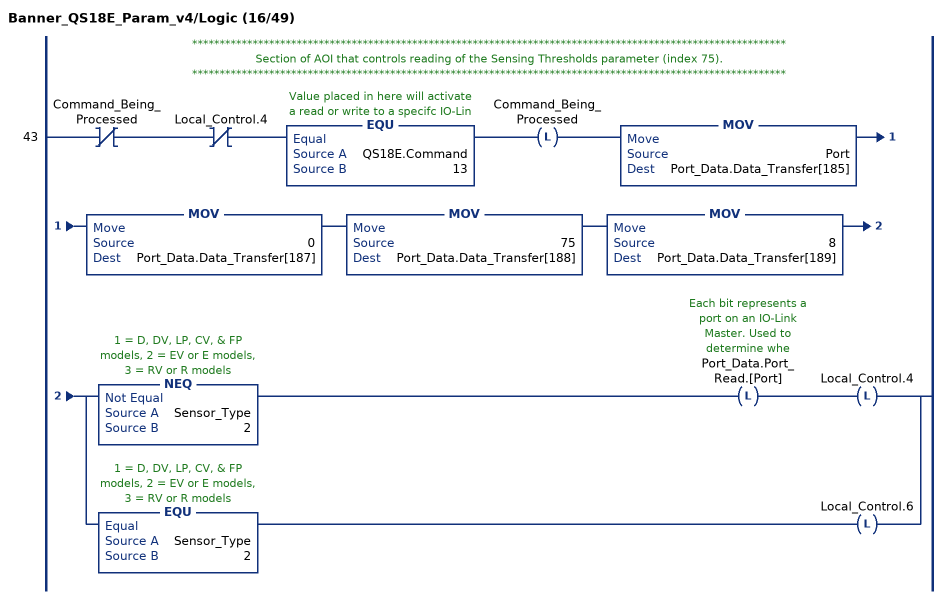
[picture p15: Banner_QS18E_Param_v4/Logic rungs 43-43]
   // ************************************************************************************************************
   // Section of AOI that controls reading of the Sensing Thresholds parameter (index 75).
   // ************************************************************************************************************
   43: XIO(Command_Being_Processed)XIO(Local_Control.4)EQU(QS18E.Command,13)OTL(Command_Being_Processed)MOV(Port,Port_Data.Data_Transfer[185])MOV(0,Port_Data.Data_Transfer[187])MOV(75,Port_Data.Data_Transfer[188])MOV(8,Port_Data.Data_Transfer[189])[NEQ(Sensor_Type,2) OTL(Port_Data.Port_Read.[Port]) OTL(Local_Control.4) ,EQU(Sensor_Type,2) OTL(Local_Control.6) ];
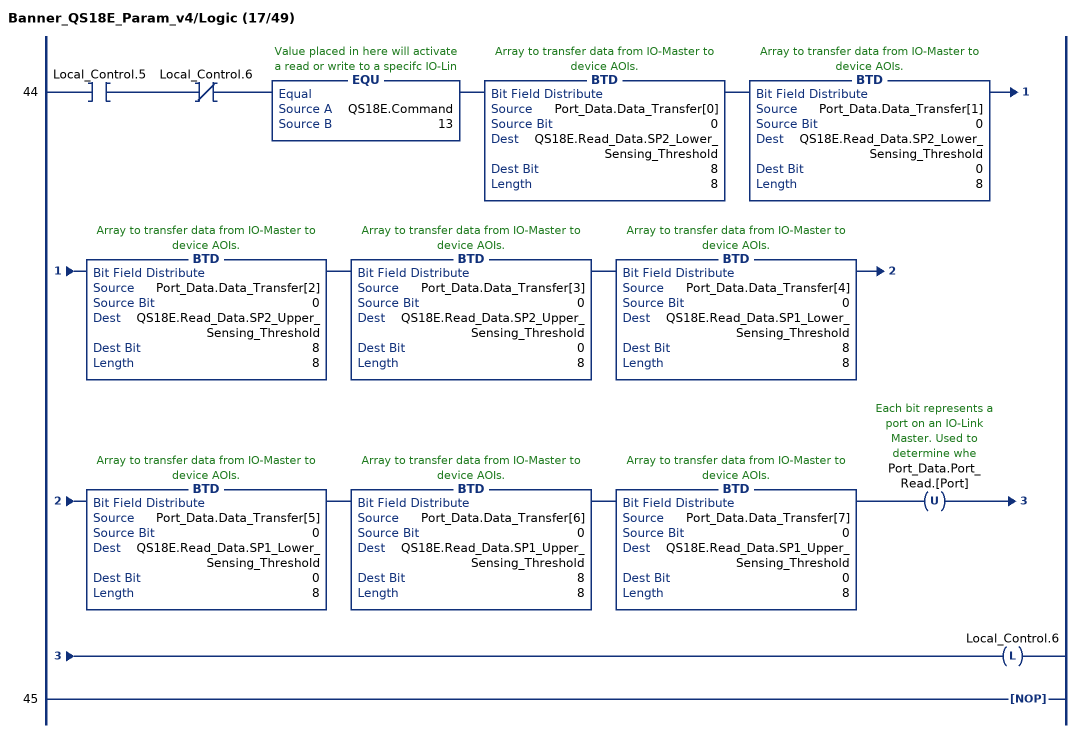
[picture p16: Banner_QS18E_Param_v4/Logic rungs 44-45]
   44: XIC(Local_Control.5)XIO(Local_Control.6)EQU(QS18E.Command,13)BTD(Port_Data.Data_Transfer[0],0,QS18E.Read_Data.SP2_Lower_Sensing_Threshold,8,8)BTD(Port_Data.Data_Transfer[1],0,QS18E.Read_Data.SP2_Lower_Sensing_Threshold,0,8)BTD(Port_Data.Data_Transfer[2],0,QS18E.Read_Data.SP2_Upper_Sensing_Threshold,8,8)BTD(Port_Data.Data_Transfer[3],0,QS18E.Read_Data.SP2_Upper_Sensing_Threshold,0,8)BTD(Port_Data.Data_Transfer[4],0,QS18E.Read_Data.SP1_Lower_Sensing_Threshold,8,8)BTD(Port_Data.Data_Transfer[5],0,QS18E.Read_Data.SP1_Lower_Sensing_Threshold,0,8)BTD(Port_Data.Data_Transfer[6],0,QS18E.Read_Data.SP1_Upper_Sensing_Threshold,8,8)BTD(Port_Data.Data_Transfer[7],0,QS18E.Read_Data.SP1_Upper_Sensing_Threshold,0,8)OTU(Port_Data.Port_Read.[Port])OTL(Local_Control.6);
   45: NOP();
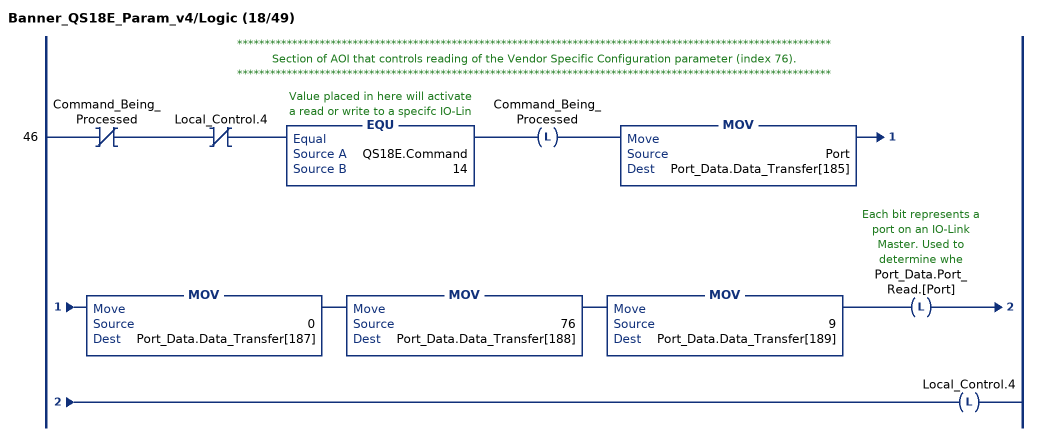
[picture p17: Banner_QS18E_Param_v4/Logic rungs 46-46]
   // ************************************************************************************************************
   // Section of AOI that controls reading of the Vendor Specific Configuration parameter (index 76).
   // ************************************************************************************************************
   46: XIO(Command_Being_Processed)XIO(Local_Control.4)EQU(QS18E.Command,14)OTL(Command_Being_Processed)MOV(Port,Port_Data.Data_Transfer[185])MOV(0,Port_Data.Data_Transfer[187])MOV(76,Port_Data.Data_Transfer[188])MOV(9,Port_Data.Data_Transfer[189])OTL(Port_Data.Port_Read.[Port])OTL(Local_Control.4);
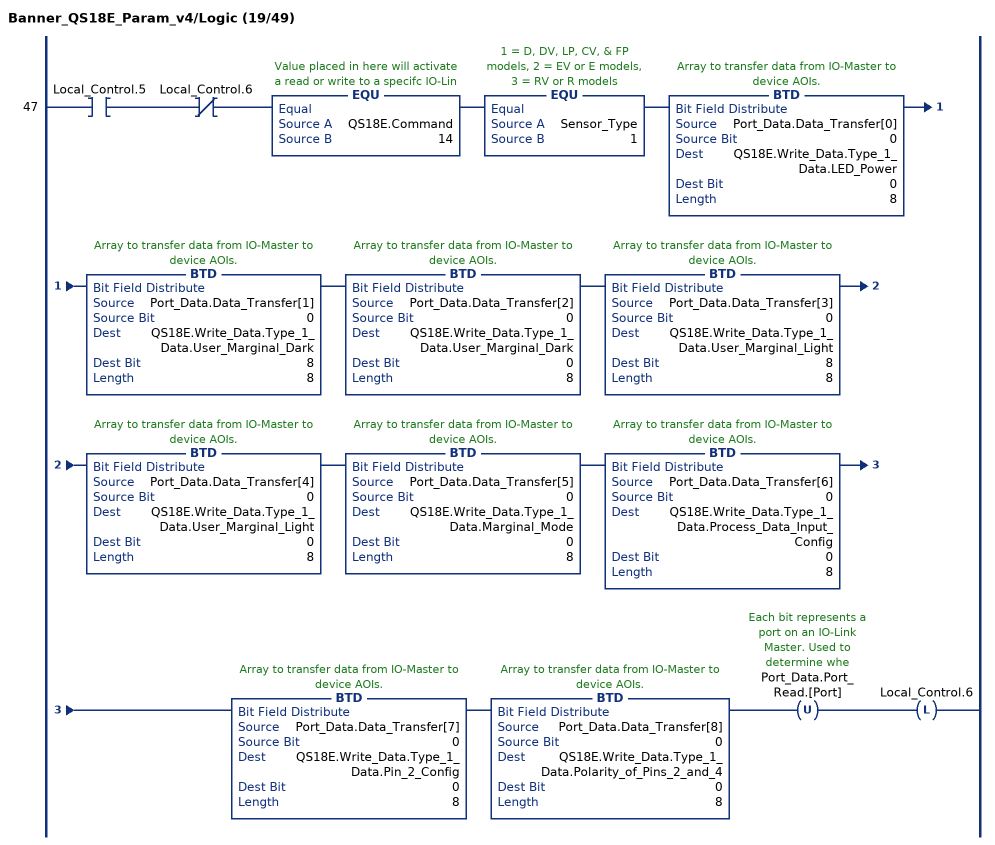
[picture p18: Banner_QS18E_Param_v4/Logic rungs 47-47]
   47: XIC(Local_Control.5)XIO(Local_Control.6)EQU(QS18E.Command,14)EQU(Sensor_Type,1)BTD(Port_Data.Data_Transfer[0],0,QS18E.Write_Data.Type_1_Data.LED_Power,0,8)BTD(Port_Data.Data_Transfer[1],0,QS18E.Write_Data.Type_1_Data.User_Marginal_Dark,8,8)BTD(Port_Data.Data_Transfer[2],0,QS18E.Write_Data.Type_1_Data.User_Marginal_Dark,0,8)BTD(Port_Data.Data_Transfer[3],0,QS18E.Write_Data.Type_1_Data.User_Marginal_Light,8,8)BTD(Port_Data.Data_Transfer[4],0,QS18E.Write_Data.Type_1_Data.User_Marginal_Light,0,8)BTD(Port_Data.Data_Transfer[5],0,QS18E.Write_Data.Type_1_Data.Marginal_Mode,0,8)BTD(Port_Data.Data_Transfer[6],0,QS18E.Write_Data.Type_1_Data.Process_Data_Input_Config,0,8)BTD(Port_Data.Data_Transfer[7],0,QS18E.Write_Data.Type_1_Data.Pin_2_Config,0,8)BTD(Port_Data.Data_Transfer[8],0,QS18E.Write_Data.Type_1_Data.Polarity_of_Pins_2_and_4,0,8)OTU(Port_Data.Port_Read.[Port])OTL(Local_Control.6);
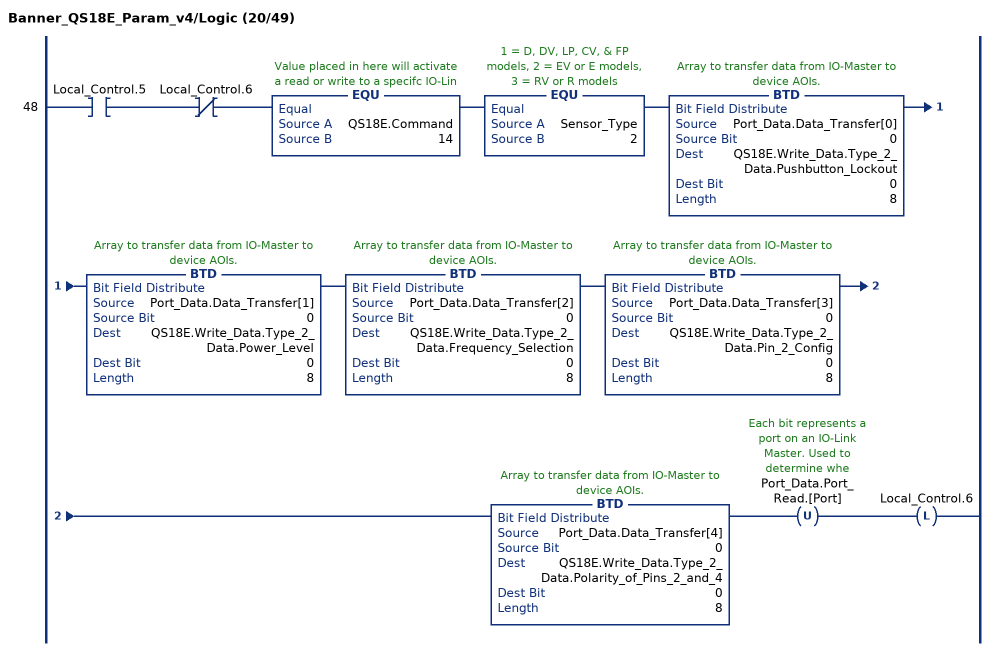
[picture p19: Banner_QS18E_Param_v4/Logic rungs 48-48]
   48: XIC(Local_Control.5)XIO(Local_Control.6)EQU(QS18E.Command,14)EQU(Sensor_Type,2)BTD(Port_Data.Data_Transfer[0],0,QS18E.Write_Data.Type_2_Data.Pushbutton_Lockout,0,8)BTD(Port_Data.Data_Transfer[1],0,QS18E.Write_Data.Type_2_Data.Power_Level,0,8)BTD(Port_Data.Data_Transfer[2],0,QS18E.Write_Data.Type_2_Data.Frequency_Selection,0,8)BTD(Port_Data.Data_Transfer[3],0,QS18E.Write_Data.Type_2_Data.Pin_2_Config,0,8)BTD(Port_Data.Data_Transfer[4],0,QS18E.Write_Data.Type_2_Data.Polarity_of_Pins_2_and_4,0,8)OTU(Port_Data.Port_Read.[Port])OTL(Local_Control.6);
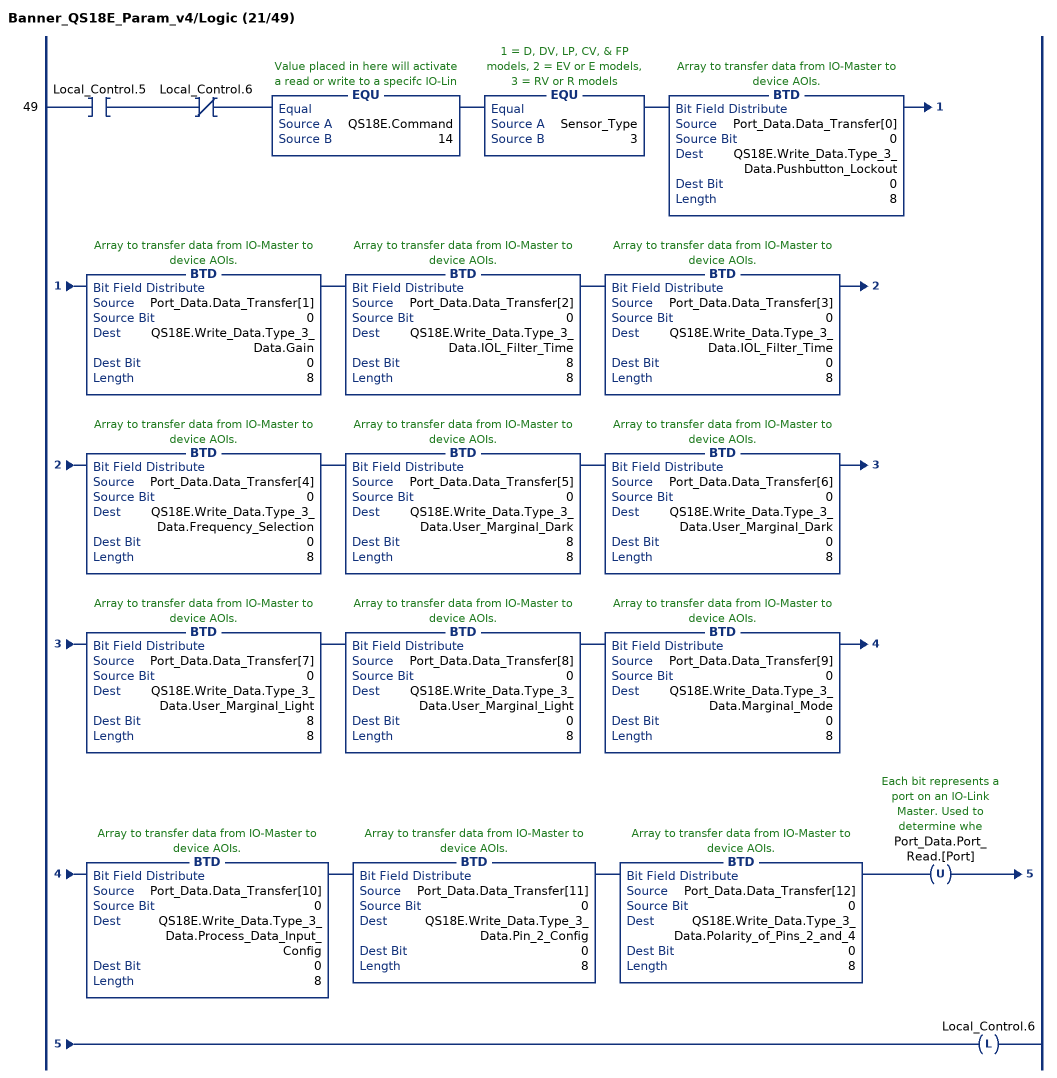
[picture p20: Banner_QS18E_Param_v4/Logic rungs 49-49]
   49: XIC(Local_Control.5)XIO(Local_Control.6)EQU(QS18E.Command,14)EQU(Sensor_Type,3)BTD(Port_Data.Data_Transfer[0],0,QS18E.Write_Data.Type_3_Data.Pushbutton_Lockout,0,8)BTD(Port_Data.Data_Transfer[1],0,QS18E.Write_Data.Type_3_Data.Gain,0,8)BTD(Port_Data.Data_Transfer[2],0,QS18E.Write_Data.Type_3_Data.IOL_Filter_Time,8,8)BTD(Port_Data.Data_Transfer[3],0,QS18E.Write_Data.Type_3_Data.IOL_Filter_Time,0,8)BTD(Port_Data.Data_Transfer[4],0,QS18E.Write_Data.Type_3_Data.Frequency_Selection,0,8)BTD(Port_Data.Data_Transfer[5],0,QS18E.Write_Data.Type_3_Data.User_Marginal_Dark,8,8)BTD(Port_Data.Data_Transfer[6],0,QS18E.Write_Data.Type_3_Data.User_Marginal_Dark,0,8)BTD(Port_Data.Data_Transfer[7],0,QS18E.Write_Data.Type_3_Data.User_Marginal_Light,8,8)BTD(Port_Data.Data_Transfer[8],0,QS18E.Write_Data.Type_3_Data.User_Marginal_Light,0,8)BTD(Port_Data.Data_Transfer[9],0,QS18E.Write_Data.Type_3_Data.Marginal_Mode,0,8)BTD(Port_Data.Data_Transfer[10],0,QS18E.Write_Data.Type_3_Data.Process_Data_Input_Config,0,8)BTD(Port_Data.Data_Transfer[11],0,QS18E.Write_Data.Type_3_Data.Pin_2_Config,0,8)BTD(Port_Data.Data_Transfer[12],0,QS18E.Write_Data.Type_3_Data.Polarity_of_Pins_2_and_4,0,8)OTU(Port_Data.Port_Read.[Port])OTL(Local_Control.6);
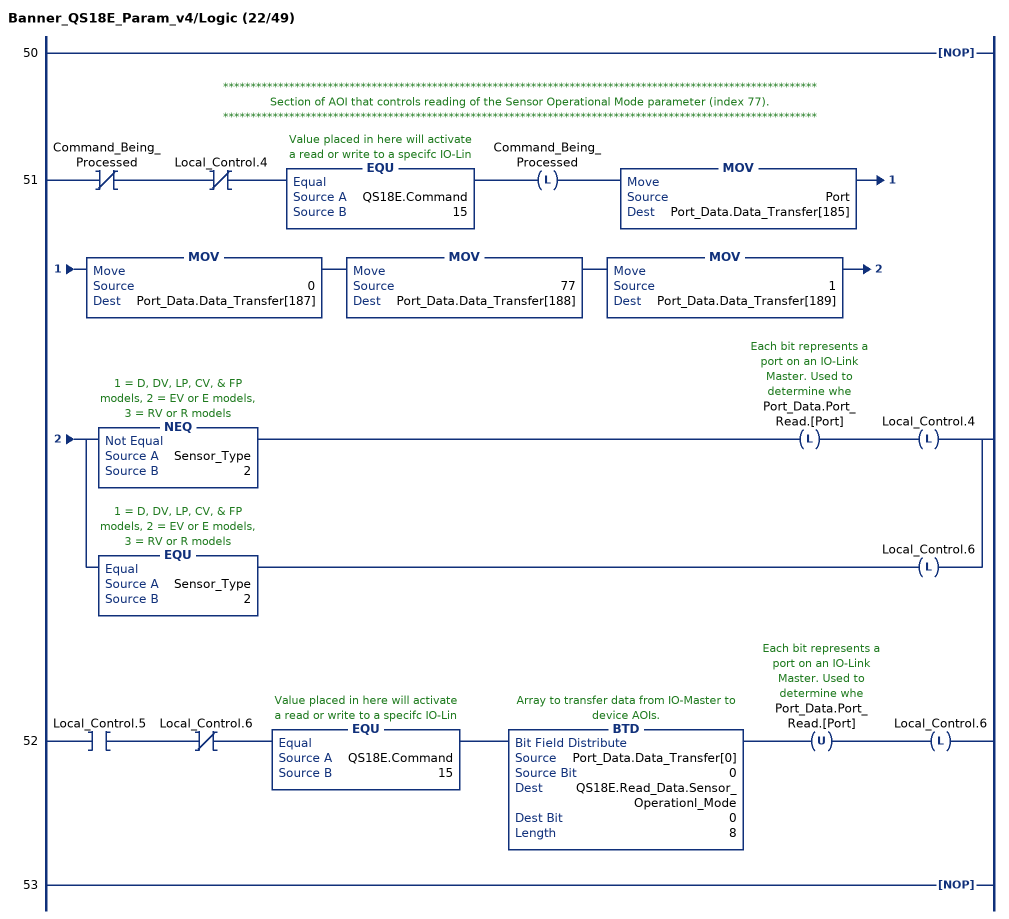
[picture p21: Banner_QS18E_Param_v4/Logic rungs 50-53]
   50: NOP();
   // ************************************************************************************************************
   // Section of AOI that controls reading of the Sensor Operational Mode parameter (index 77).
   // ************************************************************************************************************
   51: XIO(Command_Being_Processed)XIO(Local_Control.4)EQU(QS18E.Command,15)OTL(Command_Being_Processed)MOV(Port,Port_Data.Data_Transfer[185])MOV(0,Port_Data.Data_Transfer[187])MOV(77,Port_Data.Data_Transfer[188])MOV(1,Port_Data.Data_Transfer[189])[NEQ(Sensor_Type,2) OTL(Port_Data.Port_Read.[Port]) OTL(Local_Control.4) ,EQU(Sensor_Type,2) OTL(Local_Control.6) ];
   52: XIC(Local_Control.5)XIO(Local_Control.6)EQU(QS18E.Command,15)BTD(Port_Data.Data_Transfer[0],0,QS18E.Read_Data.Sensor_Operationl_Mode,0,8)OTU(Port_Data.Port_Read.[Port])OTL(Local_Control.6);
   53: NOP();
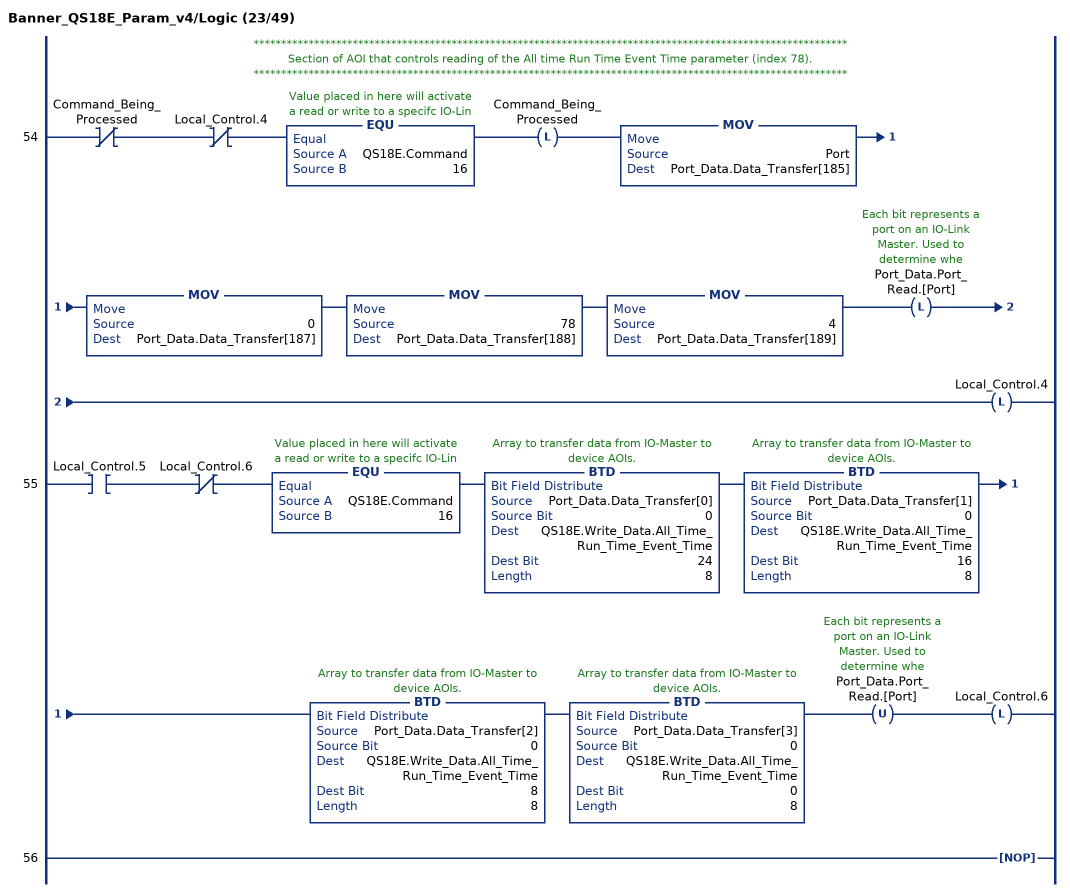
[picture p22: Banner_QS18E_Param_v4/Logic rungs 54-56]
   // ************************************************************************************************************
   // Section of AOI that controls reading of the All time Run Time Event Time parameter (index 78).
   // ************************************************************************************************************
   54: XIO(Command_Being_Processed)XIO(Local_Control.4)EQU(QS18E.Command,16)OTL(Command_Being_Processed)MOV(Port,Port_Data.Data_Transfer[185])MOV(0,Port_Data.Data_Transfer[187])MOV(78,Port_Data.Data_Transfer[188])MOV(4,Port_Data.Data_Transfer[189])OTL(Port_Data.Port_Read.[Port])OTL(Local_Control.4);
   55: XIC(Local_Control.5)XIO(Local_Control.6)EQU(QS18E.Command,16)BTD(Port_Data.Data_Transfer[0],0,QS18E.Write_Data.All_Time_Run_Time_Event_Time,24,8)BTD(Port_Data.Data_Transfer[1],0,QS18E.Write_Data.All_Time_Run_Time_Event_Time,16,8)BTD(Port_Data.Data_Transfer[2],0,QS18E.Write_Data.All_Time_Run_Time_Event_Time,8,8)BTD(Port_Data.Data_Transfer[3],0,QS18E.Write_Data.All_Time_Run_Time_Event_Time,0,8)OTU(Port_Data.Port_Read.[Port])OTL(Local_Control.6);
   56: NOP();
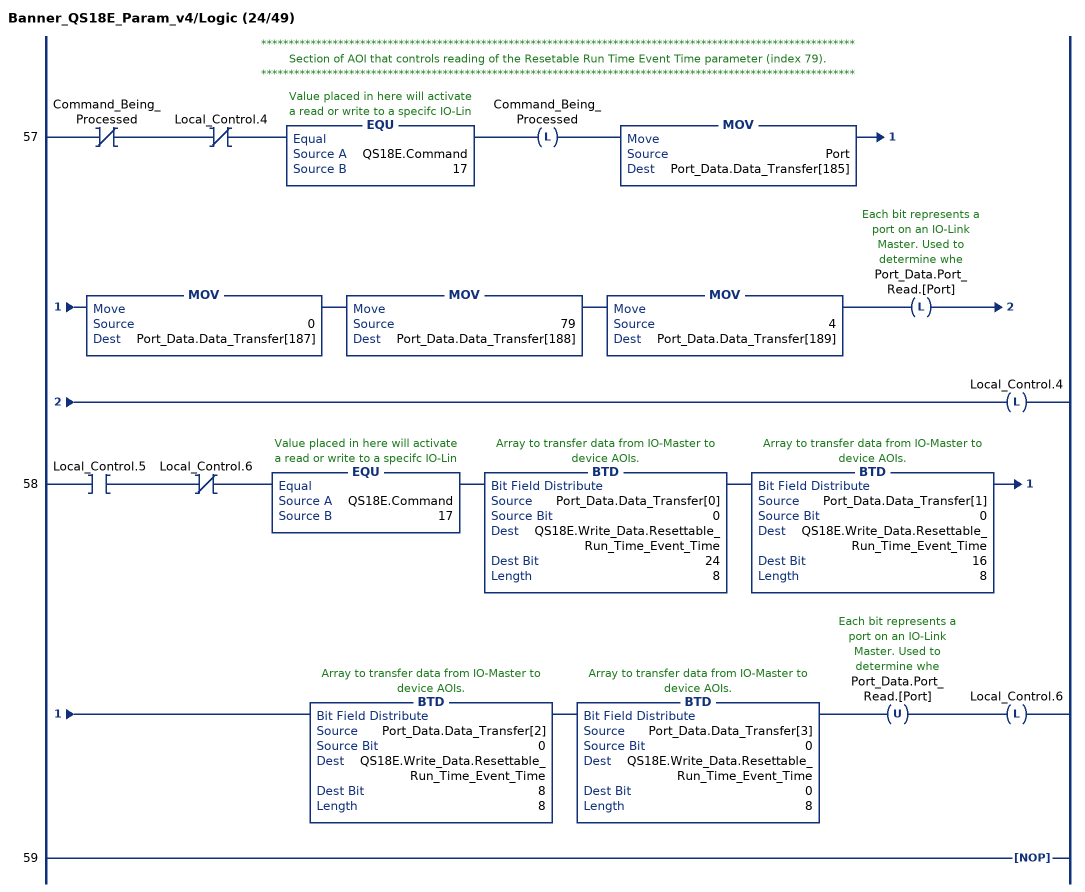
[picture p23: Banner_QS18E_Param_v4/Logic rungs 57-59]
   // ************************************************************************************************************
   // Section of AOI that controls reading of the Resetable Run Time Event Time parameter (index 79).
   // ************************************************************************************************************
   57: XIO(Command_Being_Processed)XIO(Local_Control.4)EQU(QS18E.Command,17)OTL(Command_Being_Processed)MOV(Port,Port_Data.Data_Transfer[185])MOV(0,Port_Data.Data_Transfer[187])MOV(79,Port_Data.Data_Transfer[188])MOV(4,Port_Data.Data_Transfer[189])OTL(Port_Data.Port_Read.[Port])OTL(Local_Control.4);
   58: XIC(Local_Control.5)XIO(Local_Control.6)EQU(QS18E.Command,17)BTD(Port_Data.Data_Transfer[0],0,QS18E.Write_Data.Resettable_Run_Time_Event_Time,24,8)BTD(Port_Data.Data_Transfer[1],0,QS18E.Write_Data.Resettable_Run_Time_Event_Time,16,8)BTD(Port_Data.Data_Transfer[2],0,QS18E.Write_Data.Resettable_Run_Time_Event_Time,8,8)BTD(Port_Data.Data_Transfer[3],0,QS18E.Write_Data.Resettable_Run_Time_Event_Time,0,8)OTU(Port_Data.Port_Read.[Port])OTL(Local_Control.6);
   59: NOP();
